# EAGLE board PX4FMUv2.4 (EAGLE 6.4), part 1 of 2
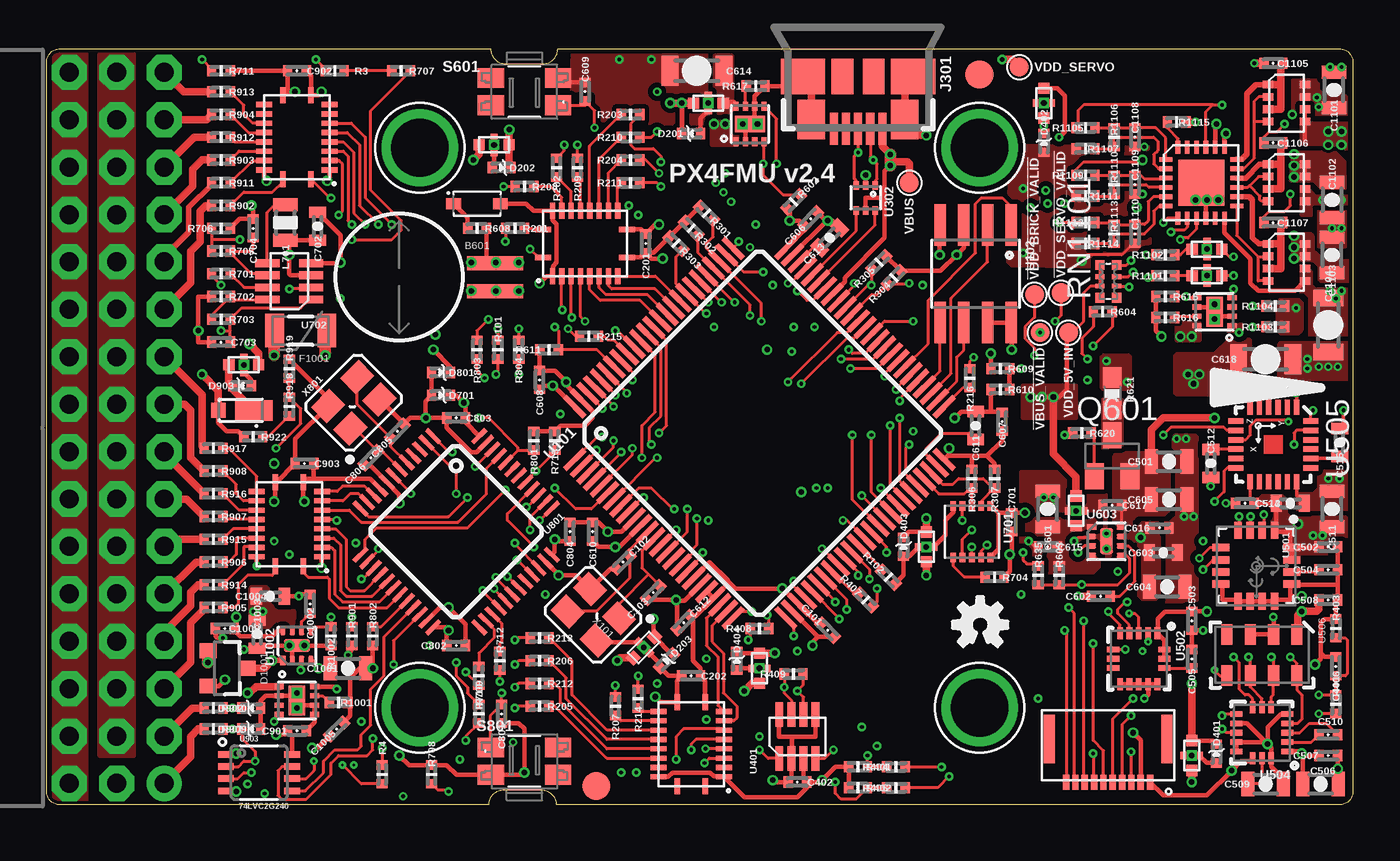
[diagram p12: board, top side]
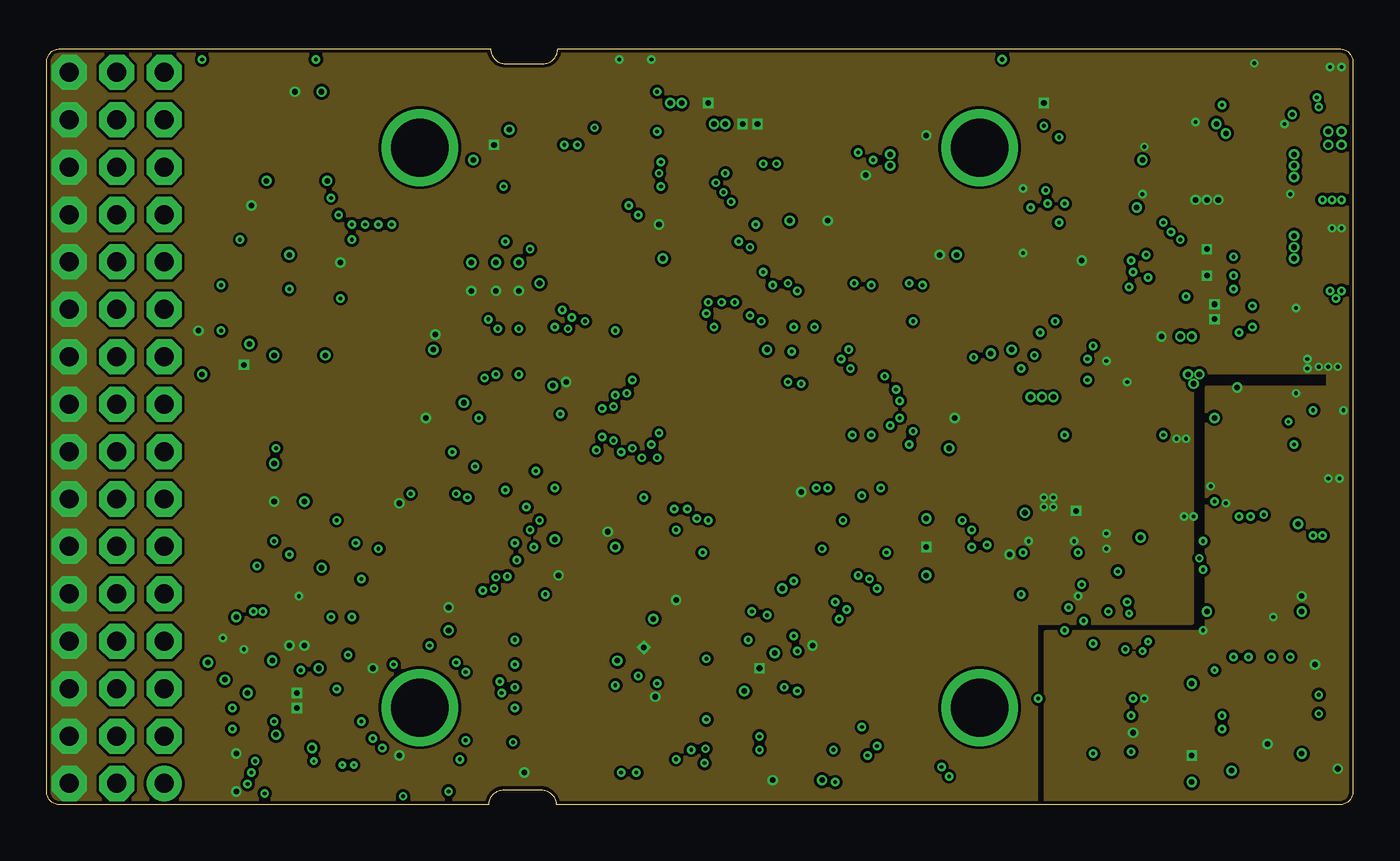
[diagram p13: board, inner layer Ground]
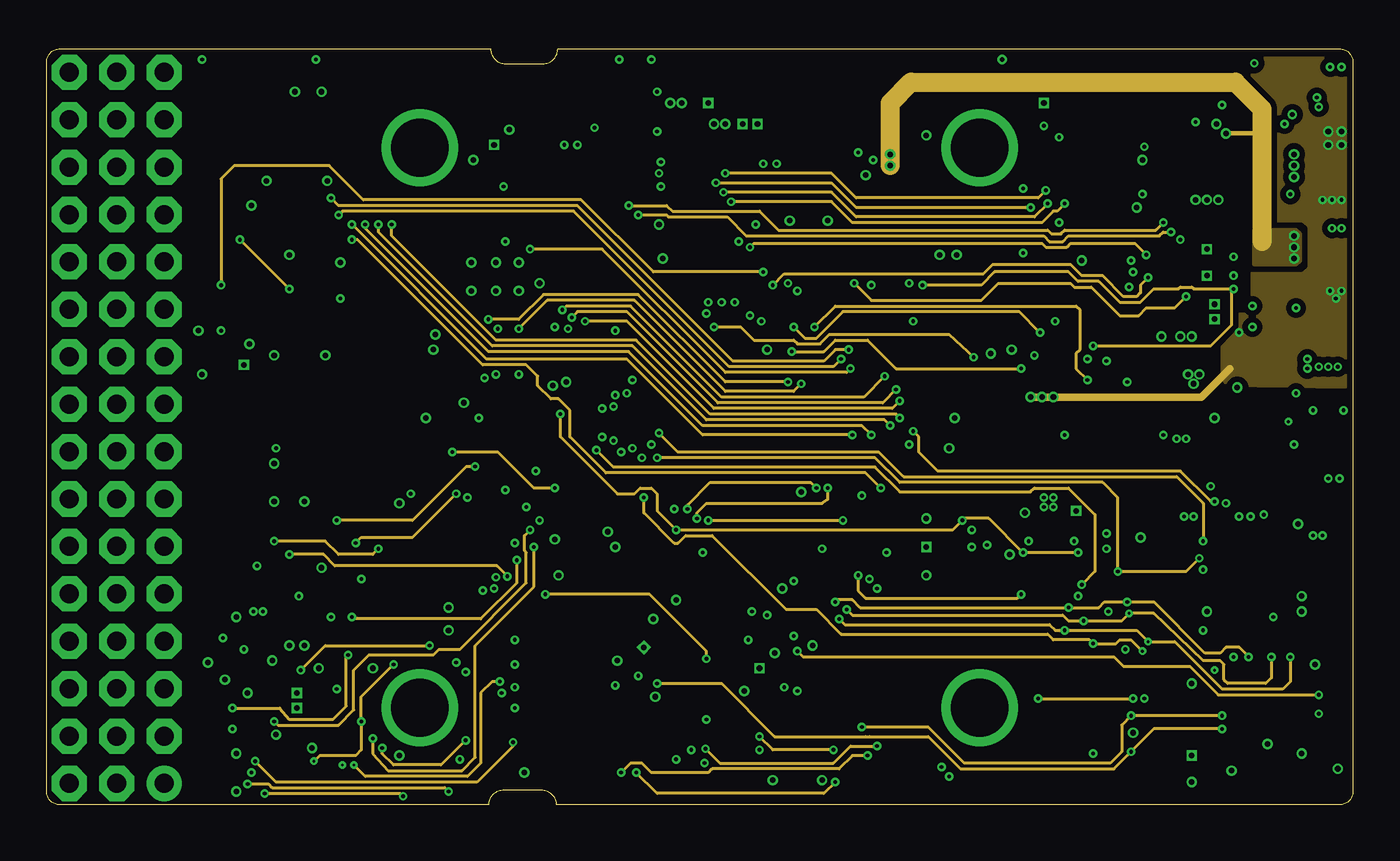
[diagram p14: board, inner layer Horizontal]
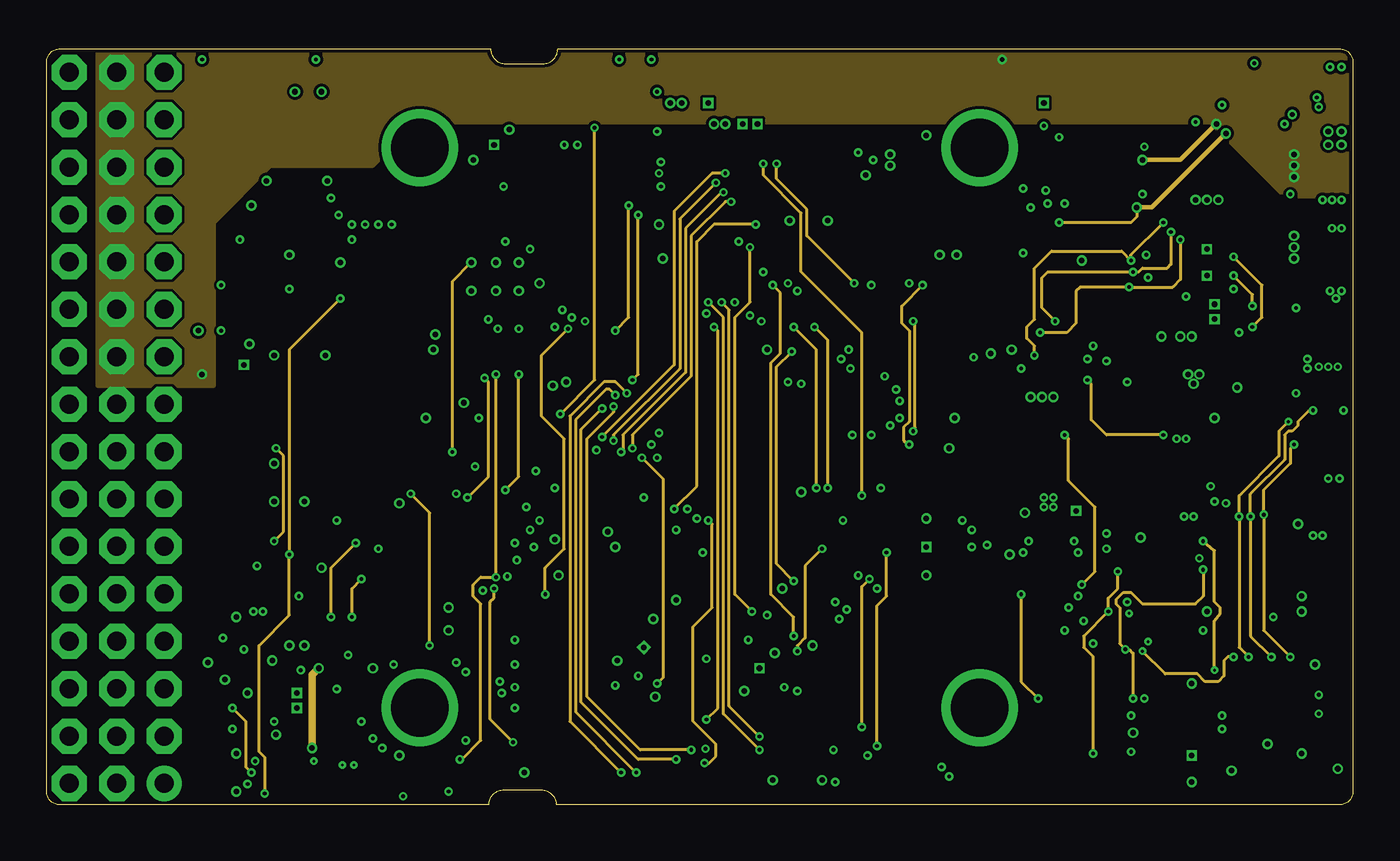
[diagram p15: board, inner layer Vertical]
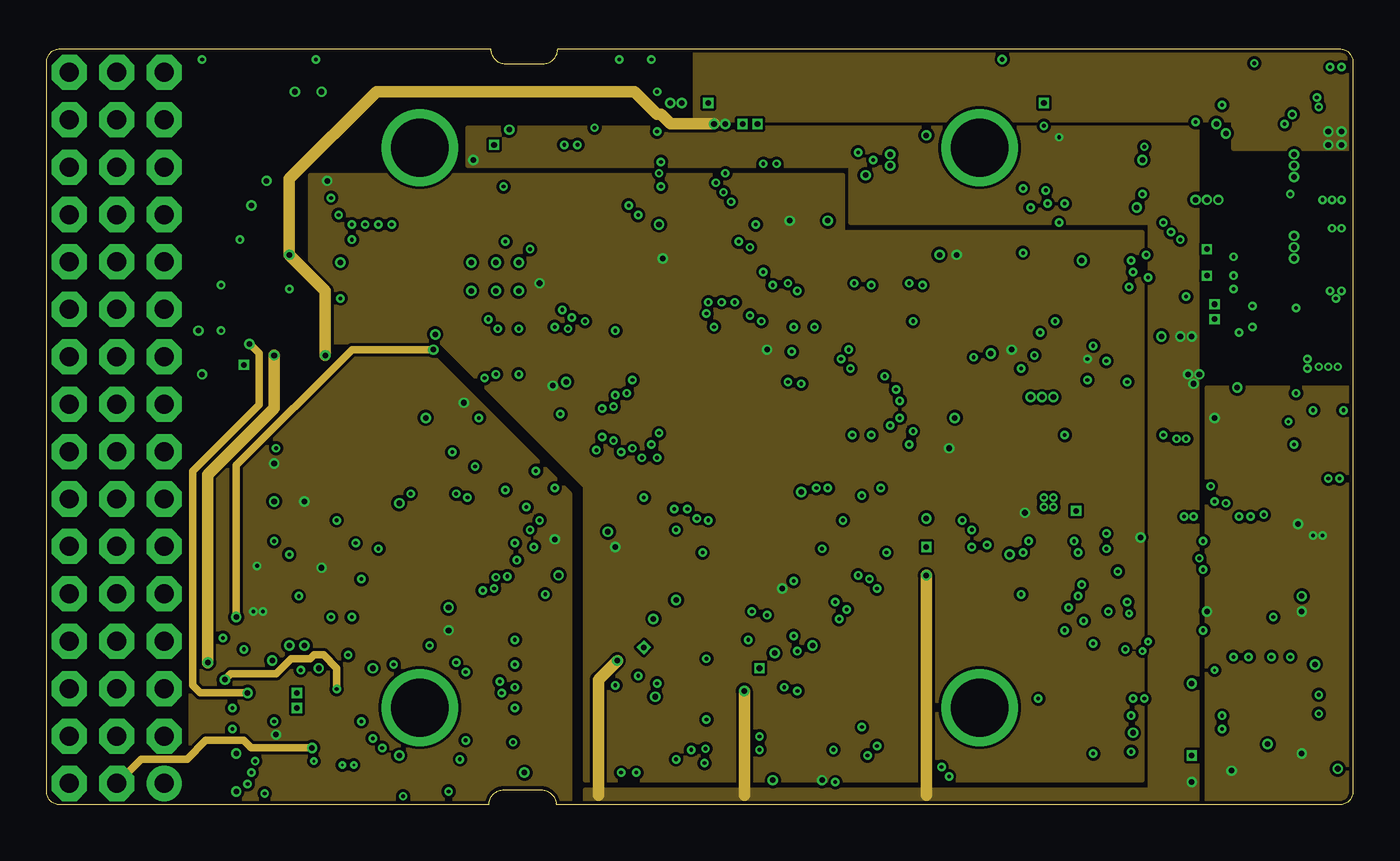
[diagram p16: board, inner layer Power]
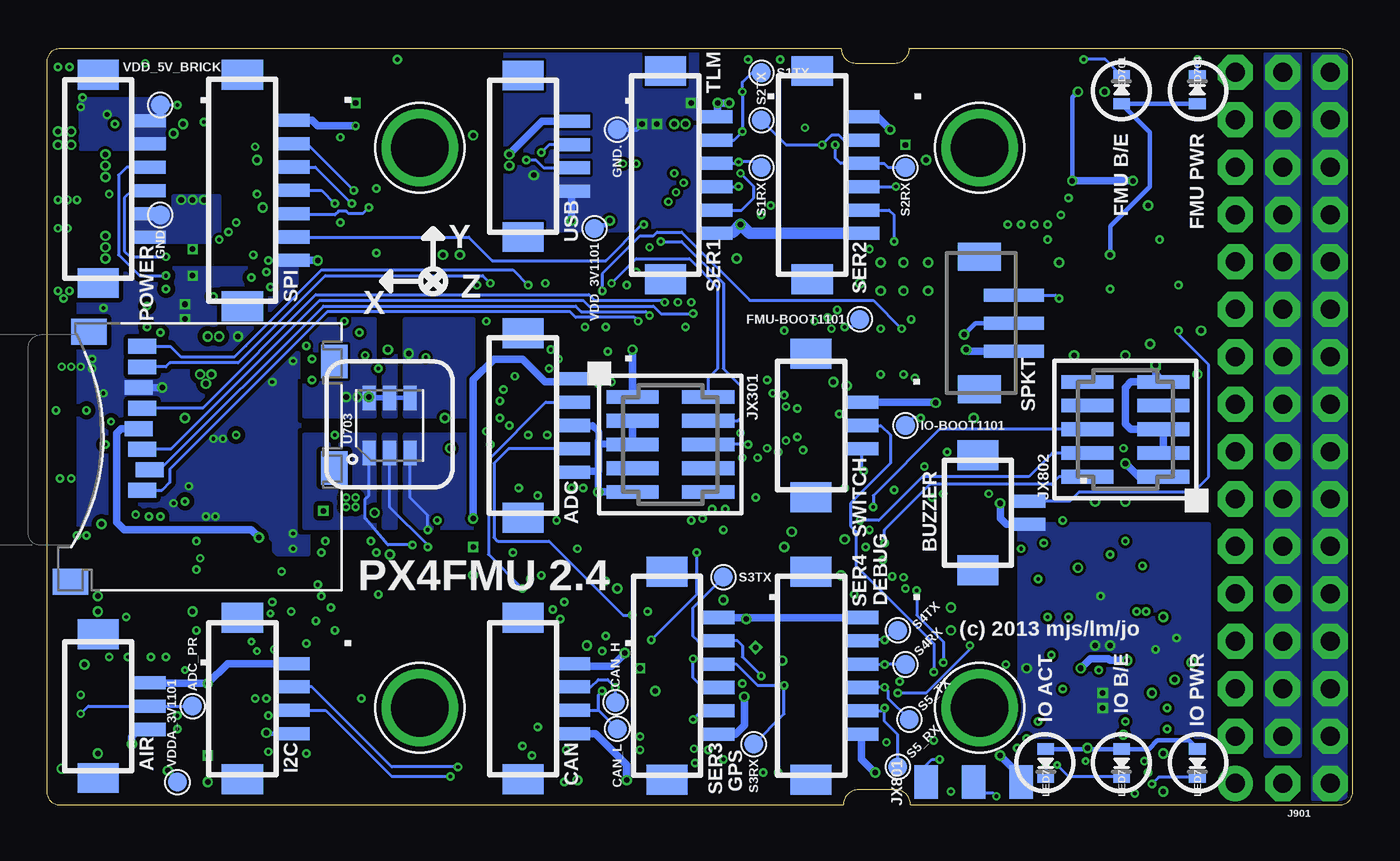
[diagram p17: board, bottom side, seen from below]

Size 70 x 40.5 mm. Coordinates in mm from the lower left corner, seen from the top.
Outline: 23.7,0 0.7,0 arc-90 0,0.7 0,39.8 arc-90 0.7,40.5 23.8,40.5 arc90 24.59,39.7 26.59,39.7 arc90 27.39,40.5 69.3,40.5 arc-90 70,39.8 70,0.7 arc-90 69.3,0 27.3,0 arc90 26.5,0.8 24.5,0.8 arc90 23.7,0
Copper layers (1*2*3*14*15*16): Top 0.035mm / dielectric 0.5mm / Ground 0.035mm / dielectric 0.15mm / Horizontal 0.035mm / dielectric 0.15mm / Vertical 0.035mm / dielectric 0.15mm / Power 0.035mm / dielectric 0.5mm / Bottom 0.035mm
Design rules "default *": minimum track width 0.15mm, minimum drill 0.2mm, track to track 5mil, track to pad 5mil, pad to pad 5mil, via to via 5mil, smd to smd 0mil, copper to edge 0.2mm, drill to drill 0.2mm, minimum pad ring 0.125mm, minimum via ring 0.125mm, stop-mask expansion 1mil, vias tented up to drill 0.31mm, thermal gap 8mil
Net classes: 0 signal: width 0.15 mm, drill 0.15 mm, clearance 0.152 mm; 1 power: width 0.15 mm, drill 0.2 mm, clearance 0.152 mm

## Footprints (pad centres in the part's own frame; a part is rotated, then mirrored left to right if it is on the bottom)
PAD.04X.04 = smd 1.016 x 1.016: P$1 0,0
MS621FE = smd 3 x 0.75: 1 5.15,0.75; 2 5.15,-0.75
0402-CAP = smd 0.5 x 0.6: P$1 -0.5,0; P$2 0.5,0
0805-CAP = smd 0.7 x 1.3: P$1 -0.95,0; P$2 0.95,0
0603-CAP = smd 0.6 x 0.9: P$1 -0.75,0; P$2 0.75,0
1206-CAP = smd 0.9 x 1.6: P$1 -1.45,0; P$2 1.45,0
MICROSMP = smd 0.8 x 0.8: ANODE 0.65,0 | smd 2 x 1.1: CATHODE -1.25,0
SOD323 = smd 0.8 x 0.6: A 1.25,0; C -1.25,0
0402-TVS = smd 0.5 x 0.6: A 0.5,0; C -0.5,0
SOT23-3 = smd 0.8 x 0.9: 1 -0.95,-1; 2 0.95,-1; 3 0,1.1
PTC-1206 = smd 1 x 1.8: 1 -1.4,0; 2 1.4,0
DF13C-6P-1.25V = smd 0.7 x 1.8: 1 -3.125,0.9; 2 -1.875,0.9; 3 -0.625,0.9; 4 0.625,0.9; 5 1.875,0.9; 6 3.125,0.9 | smd 1.6 x 2.2: M$0 5.575,-1.8; M$1 -5.575,-1.8
MOLEX-47346-0001 = smd 1.7 x 0.44: D+ 2.8,0; D- 2.8,0.65; GND 2.8,-1.3; ID 2.8,-0.65; VBUS 2.8,1.3 | smd 1.9 x 2.375: GND1 0,2.95; GND4 0,-2.95 | smd 2.1 x 1.475: GND2 2.3,2.5; GND3 2.3,-2.5 | smd 1.9 x 1.175: GND5 0,-0.838; GND6 0,0.838
DF13C-4P-1.25V = smd 0.7 x 1.8: 1 -1.875,0.9; 2 -0.625,0.9; 3 0.625,0.9; 4 1.875,0.9 | smd 1.6 x 2.2: M$0 4.325,-1.8; M$1 -4.325,-1.8
DF13C-3P-1.25V = smd 0.7 x 1.8: 1 -1.25,0.9; 2 0,0.9; 3 1.25,0.9 | smd 1.6 x 2.2: M$0 3.85,-1.8; M$1 -3.85,-1.8
DF13C-7P-1.25V = smd 0.7 x 1.8: 1 -3.75,0.9; 2 -2.5,0.9; 3 -1.25,0.9; 4 0,0.9; 5 1.25,0.9; 6 2.5,0.9; 7 3.75,0.9 | smd 1.6 x 2.2: M$0 6.2,-1.8; M$1 -6.2,-1.8
DF13C-5P-1.25V = smd 0.7 x 1.8: 1 -2.5,0.9; 2 -1.25,0.9; 3 0,0.9; 4 1.25,0.9; 5 2.5,0.9 | smd 1.6 x 2.2: M$0 4.95,-1.8; M$1 -4.95,-1.8
DF13C-2P-1.25V = smd 0.7 x 1.8: 1 -0.625,0.9; 2 0.625,0.9 | smd 1.6 x 2.2: M$0 3.075,-1.8; M$1 -3.075,-1.8
JST-ZH-SMT-VERTICAL = smd 0.7 x 3.2: P$1 -1.5,-1.75; P$2 0,-1.75; P$3 1.5,-1.75 | smd 1.5 x 2.3: P$4 3.55,0.1; P$5 -3.55,0.1
3X16RA = drill 1.016 pad 1.88: 1 2.54,19.05 | drill 1.016 pad 1.88 octagon: 2 0,19.05; 3 -2.54,19.05; 4 2.54,16.51; 5 0,16.51; 6 -2.54,16.51; 7 2.54,13.97; 8 0,13.97; 9 -2.54,13.97; 10 2.54,11.43; 11 0,11.43; 12 -2.54,11.43; 13 2.54,8.89; 14 0,8.89; 15 -2.54,8.89; 16 2.54,6.35; 17 0,6.35; 18 -2.54,6.35; 19 2.54,3.81; 20 0,3.81; 21 -2.54,3.81; 22 2.54,1.27; 23 0,1.27; 24 -2.54,1.27; 25 2.54,-1.27; 26 0,-1.27; 27 -2.54,-1.27; 28 2.54,-3.81; 29 0,-3.81; 30 -2.54,-3.81; 31 2.54,-6.35; 32 0,-6.35; 33 -2.54,-6.35; 34 2.54,-8.89; 35 0,-8.89; 36 -2.54,-8.89; 37 2.54,-11.43; 38 0,-11.43; 39 -2.54,-11.43; 40 2.54,-13.97; 41 0,-13.97; 42 -2.54,-13.97; 43 2.54,-16.51; 44 0,-16.51; 45 -2.54,-16.51; 46 2.54,-19.05; 47 0,-19.05; 48 -2.54,-19.05
FIDUCIAL-1.5X3 = smd 1.5 x 1.5: 1 0,0
FTSH-105-01-XXX-DV-K = smd 0.737 x 2.794: 1 -2.54,-2.032; 2 -2.54,2.032; 3 -1.27,-2.032; 4 -1.27,2.032; 5 0,-2.032; 6 0,2.032; 7 1.27,-2.032; 8 1.27,2.032; 9 2.54,-2.032; 10 2.54,2.032
HEADER_3X01_SMD_H_BOARD_EDGE_SHORT = smd 1.27 x 1.778: 1 -2.54,0; 2 0,0; 3 2.54,0
KYOCERA-KNH16-DA = smd 0.6 x 0.6: P$1 -0.8,0; P$2 0.8,0 | smd 0.4 x 0.4: P$3 0,-0.4; P$4 0,0.4 | drill 0.3 pad 0.4 square: P$5 0,0
0805-IND = smd 0.7 x 1.3: P$1 -0.95,0; P$2 0.95,0
0603-LED = smd 0.6 x 0.9: A 0.75,0; C -0.75,0
MOUNT-HOLE3.1 = drill 3.1 pad 4.1: P$1 0,0
SOT23-BEC = smd 1 x 1.4: B -0.95,-1.1; C 0,1.1; E 0.95,-1.1
0402-RES = smd 0.5 x 0.6: P$1 -0.5,0; P$2 0.5,0
0603-RES = smd 1.1 x 1: 1 -0.85,0; 2 0.85,0
EXB28V = smd 0.525 x 0.5: 1 -0.875,-0.45; 4 0.875,-0.45; 5 0.875,0.45; 8 -0.875,0.45 | smd 0.25 x 0.5: 2 -0.25,-0.45; 3 0.25,-0.45; 6 0.25,0.45; 7 -0.25,0.45
EVQP7J01K = smd 1.4 x 1.05: A1 -1.8,0.725; A2 1.8,0.725; B3 -1.8,-0.725; B4 1.8,-0.725
TQFP100 = smd 1.5 x 0.29: 1 -8,6; 2 -8,5.5; 3 -8,5; 4 -8,4.5; 5 -8,4; 6 -8,3.5; 7 -8,3; 8 -8,2.5; 9 -8,2; 10 -8,1.5; 11 -8,1; 12 -8,0.5; 13 -8,0; 14 -8,-0.5; 15 -8,-1; 16 -8,-1.5; 17 -8,-2; 18 -8,-2.5; 19 -8,-3; 20 -8,-3.5; 21 -8,-4; 22 -8,-4.5; 23 -8,-5; 24 -8,-5.5; 25 -8,-6; 51 8,-6; 52 8,-5.5; 53 8,-5; 54 8,-4.5; 55 8,-4; 56 8,-3.5; 57 8,-3; 58 8,-2.5; 59 8,-2; 60 8,-1.5; 61 8,-1; 62 8,-0.5; 63 8,0; 64 8,0.5; 65 8,1; 66 8,1.5; 67 8,2; 68 8,2.5; 69 8,3; 70 8,3.5; 71 8,4; 72 8,4.5; 73 8,5; 74 8,5.5; 75 8,6 | smd 0.29 x 1.5: 26 -6,-8; 27 -5.5,-8; 28 -5,-8; 29 -4.5,-8; 30 -4,-8; 31 -3.5,-8; 32 -3,-8; 33 -2.5,-8; 34 -2,-8; 35 -1.5,-8; 36 -1,-8; 37 -0.5,-8; 38 0,-8; 39 0.5,-8; 40 1,-8; 41 1.5,-8; 42 2,-8; 43 2.5,-8; 44 3,-8; 45 3.5,-8; 46 4,-8; 47 4.5,-8; 48 5,-8; 49 5.5,-8; 50 6,-8; 76 6,8; 77 5.5,8; 78 5,8; 79 4.5,8; 80 4,8; 81 3.5,8; 82 3,8; 83 2.5,8; 84 2,8; 85 1.5,8; 86 1,8; 87 0.5,8; 88 0,8; 89 -0.5,8; 90 -1,8; 91 -1.5,8; 92 -2,8; 93 -2.5,8; 94 -3,8; 95 -3.5,8; 96 -4,8; 97 -4.5,8; 98 -5,8; 99 -5.5,8; 100 -6,8
SO08 = smd 0.61 x 2.21: 1 -1.905,-2.616; 2 -0.635,-2.616; 3 0.635,-2.616; 4 1.905,-2.616; 5 1.905,2.616; 6 0.635,2.616; 7 -0.635,2.616; 8 -1.905,2.616
QFN20-RGY = smd 0.28 x 0.85: 1 -0.75,2.25; 10 -0.75,-2.25; 11 0.75,-2.25; 20 0.75,2.25 | smd 0.85 x 0.28: 2 -1.75,1.75; 3 -1.75,1.25; 4 -1.75,0.75; 5 -1.75,0.25; 6 -1.75,-0.25; 7 -1.75,-0.75; 8 -1.75,-1.25; 9 -1.75,-1.75; 12 1.75,-1.75; 13 1.75,-1.25; 14 1.75,-0.75; 15 1.75,-0.25; 16 1.75,0.25; 17 1.75,0.75; 18 1.75,1.25; 19 1.75,1.75
MICROSD = smd 0.8 x 1.5: 1 -1.94,2.7; 2 -0.84,2.3; 3 0.26,2.7; 4 1.36,2.9; 5 2.46,2.7; 6 3.56,2.9; 7 4.66,2.7; 8 5.76,2.7 | smd 1.4 x 1.9: NC -6.85,6.55; NC3 6.55,5.55 | smd 1.8 x 1.4: NC1 -0.75,-7.6; NC2 4.95,-7.6
SOT563-6 = smd 0.3 x 0.45: 1 -0.5,-0.675; 2 0,-0.675; 3 0.5,-0.675; 4 0.5,0.675; 5 0,0.675; 6 -0.5,0.675
SOT23-8 = smd 0.42 x 1.3: 1 -0.975,-1.175; 2 -0.325,-1.175; 3 0.325,-1.175; 4 0.975,-1.175; 5 0.975,1.175; 6 0.325,1.175; 7 -0.325,1.175; 8 -0.975,1.175
L3G4200DH-MAN = smd 0.9 x 0.4: 1 -1.9,0.975; 2 -1.9,0.325; 3 -1.9,-0.325; 4 -1.9,-0.975; 9 1.9,-0.975; 10 1.9,-0.325; 11 1.9,0.325; 12 1.9,0.975 | smd 0.4 x 0.9: 5 -0.975,-1.9; 6 -0.325,-1.9; 7 0.325,-1.9; 8 0.975,-1.9; 13 0.975,1.9; 14 0.325,1.9; 15 -0.325,1.9; 16 -0.975,1.9
LGA-16L = smd 0.65 x 0.3: 1 -1.37,1; 2 -1.37,0.5; 3 -1.37,0; 4 -1.37,-0.5; 5 -1.37,-1; 9 1.37,-1; 10 1.37,-0.5; 11 1.37,0; 12 1.37,0.5; 13 1.37,1 | smd 0.3 x 0.65: 6 -0.5,-1.37; 7 0,-1.37; 8 0.5,-1.37; 14 0.5,1.37; 15 0,1.37; 16 -0.5,1.37
QFN-24 = smd 0.8 x 0.29: 1 -2,1.25; 2 -2,0.75; 3 -2,0.25; 4 -2,-0.25; 5 -2,-0.75; 6 -2,-1.25; 13 2,-1.25; 14 2,-0.75; 15 2,-0.25; 16 2,0.25; 17 2,0.75; 18 2,1.25 | smd 0.29 x 0.8: 7 -1.25,-2; 8 -0.75,-2; 9 -0.25,-2; 10 0.25,-2; 11 0.75,-2; 12 1.25,-2; 19 1.25,2; 20 0.75,2; 21 0.25,2; 22 -0.25,2; 23 -0.75,2; 24 -1.25,2
MS5611-01BA = smd 1.1 x 0.6: 1 -1.1,1.875; 2 -1.1,0.625; 3 -1.1,-0.625; 4 -1.1,-1.875; 5 1.1,-1.875; 6 1.1,-0.625; 7 1.1,0.625; 8 1.1,1.875
QFN8-DSG = smd 0.28 x 0.5: 1 -0.75,-0.95; 2 -0.25,-0.95; 3 0.25,-0.95; 4 0.75,-0.95; 5 0.75,0.95; 6 0.25,0.95; 7 -0.25,0.95; 8 -0.75,0.95 | smd 1.6 x 0.9: GND 0,0 | drill 0.3 square: P$2 -0.4,0; P$3 0.4,0
MLF-8-EPAD = smd 0.5 x 0.3: 1 -0.8,0.75; 2 -0.8,0.25; 3 -0.8,-0.25; 4 -0.8,-0.75; 5 0.8,-0.75; 6 0.8,-0.25; 7 0.8,0.25; 8 0.8,0.75 | smd 0.7 x 1.4: GND 0,0
SON10 = smd 0.32 x 0.5: 1 -1,-1.375; 2 -0.5,-1.375; 3 0,-1.375; 4 0.5,-1.375; 5 1,-1.375; 6 1,1.375; 7 0.5,1.375; 8 0,1.375; 9 -0.5,1.375; 10 -1,1.375
6-PLCC = smd 1.3 x 0.7: A1 1.475,1.1; A2 1.475,0; A3 1.475,-1.1; C1 -1.475,1.1; C2 -1.475,0; C3 -1.475,-1.1
TQFP48 = smd 0.24 x 1: 1 -2.75,-4.5; 2 -2.25,-4.5; 3 -1.75,-4.5; 4 -1.25,-4.5; 5 -0.75,-4.5; 6 -0.25,-4.5; 7 0.25,-4.5; 8 0.75,-4.5; 9 1.25,-4.5; 10 1.75,-4.5; 11 2.25,-4.5; 12 2.75,-4.5; 25 2.75,4.5; 26 2.25,4.5; 27 1.75,4.5; 28 1.25,4.5; 29 0.75,4.5; 30 0.25,4.5; 31 -0.25,4.5; 32 -0.75,4.5; 33 -1.25,4.5; 34 -1.75,4.5; 35 -2.25,4.5; 36 -2.75,4.5 | smd 1 x 0.24: 13 4.5,-2.75; 14 4.5,-2.25; 15 4.5,-1.75; 16 4.5,-1.25; 17 4.5,-0.75; 18 4.5,-0.25; 19 4.5,0.25; 20 4.5,0.75; 21 4.5,1.25; 22 4.5,1.75; 23 4.5,2.25; 24 4.5,2.75; 37 -4.5,2.75; 38 -4.5,2.25; 39 -4.5,1.75; 40 -4.5,1.25; 41 -4.5,0.75; 42 -4.5,0.25; 43 -4.5,-0.25; 44 -4.5,-0.75; 45 -4.5,-1.25; 46 -4.5,-1.75; 47 -4.5,-2.25; 48 -4.5,-2.75
TSSOP8_SOT505-2 = smd 0.35 x 0.85: 1 -0.975,-1.775; 2 -0.325,-1.775; 3 0.325,-1.775; 4 0.975,-1.775; 5 0.975,1.775; 6 0.325,1.775; 7 -0.325,1.775; 8 -0.975,1.775
MO-220 = smd 0.7 x 0.25: P$1 -1.9,1.25; P$2 -1.9,0.75; P$3 -1.9,0.25; P$4 -1.9,-0.25; P$5 -1.9,-0.75; P$6 -1.9,-1.25; P$13 1.9,-1.25; P$14 1.9,-0.75; P$15 1.9,-0.25; P$16 1.9,0.25; P$17 1.9,0.75; P$18 1.9,1.25 | smd 0.25 x 0.7: P$7 -1.25,-1.9; P$8 -0.75,-1.9; P$9 -0.25,-1.9; P$10 0.25,-1.9; P$11 0.75,-1.9; P$12 1.25,-1.9; P$19 1.25,1.9; P$20 0.75,1.9; P$21 0.25,1.9; P$22 -0.25,1.9; P$23 -0.75,1.9; P$24 -1.25,1.9 | smd 2.45 x 2.45: P$25 0,0
1206-8 = smd 0.406 x 0.559: P$1 -0.991,-0.991; P$2 -0.33,-0.991; P$3 0.33,-0.991; P$4 0.991,-0.991; P$5 0.991,0.991; P$6 0.33,0.991; P$7 -0.33,0.991; P$8 -0.991,0.991
OSCILLATOR-3.2X2.5 = smd 1.4 x 1.2: 1 -1.1,-0.85; 2 1.1,-0.85; 3 1.1,0.85; 4 -1.1,0.85
51281-1094 = smd 0.34 x 0.8: 1 0,0; 2 0.5,0; 3 1,0; 4 1.5,0; 5 2,0; 6 2.5,0; 7 3,0; 8 3.5,0; 9 4,0; 10 4.5,0 | smd 0.6 x 2.6: P$11 -0.9,-2.3; P$12 5.4,-2.3

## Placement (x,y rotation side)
!VBUS_VALID  PAD.04  [PAD.04X.04]  53.24,25.3 270 top
!VDD_BRICK_VALID  PAD.04  [PAD.04X.04]  52.93,27.33 90 top
!VDD_SERVO_VALID  PAD.04  [PAD.04X.04]  54.36,27.43 90 top
ADC_PR  PAD.04  [PAD.04X.04]  62.18,5.28 270 bottom
B601  MS621FE  [MS621FE]  18.89,28.27 0 top
C101  0u1  [0402-CAP]  41.86,9.35 315 top
C102  8p  [0402-CAP]  30.89,13 225 top
C103  8p  [0402-CAP]  32.51,11.38 45 top
C201  0u1  [0402-CAP]  32.11,30.07 90 top
C202  0u1  [0402-CAP]  34.54,6.91 180 top
C401  0u1  [0402-CAP]  69.09,7.42 90 top
C402  0u1  [0402-CAP]  40.23,1.22 180 top
C501  10u/10V  [0805-CAP]  60.15,18.39 0 top
C502  0u1  [0402-CAP]  68.68,13.82 0 top
C503  0u1  [0402-CAP]  61.37,9.86 270 top
C504  10n  [0402-CAP]  68.68,12.6 0 top
C505  10n  [0402-CAP]  61.37,7.82 90 top
C506  10u/10V  [0805-CAP]  68.28,1.12 0 top
C507  0u1  [0402-CAP]  68.68,2.64 0 top
C508  0u1  [0402-CAP]  68.68,10.97 0 top
C509  10u/10V  [0805-CAP]  65.33,1.12 0 top
C510  0u47  [0402-CAP]  68.68,3.76 0 top
C511  10u/10V  [0805-CAP]  68.88,15.85 90 top
C512  2u2  [0603-CAP]  62.38,18.29 270 top
C513  2u2  [0603-CAP]  66.65,16.15 0 top
C514  0u1  [0402-CAP]  64.21,16.15 180 top
C515  0u01  [0603-CAP]  69.29,19.41 90 top
C601  10u/25V  [0805-CAP]  53.64,15.85 90 top
C602  10n  [0402-CAP]  56.49,11.18 0 top
C603  1u  [0603-CAP]  59.84,13.51 0 top
C604  22u/25V  [0805-CAP]  60.05,11.68 0 top
C605  22u/25V  [0805-CAP]  60.15,16.36 0 top
C606  0u1  [0402-CAP]  40.94,31.39 45 top
C607  0u1  [0402-CAP]  51.21,20.52 90 top
C608  0u1  [0402-CAP]  26.42,22.76 90 top
C609  0u1  [0402-CAP]  28.85,38.2 270 top
C610  0u1  [0402-CAP]  29.26,14.63 90 top
C611  2u2  [0603-CAP]  49.78,20.32 90 top
C612  0u1  [0402-CAP]  34.14,9.75 225 top
C613  2u2  [0603-CAP]  41.96,30.38 45 top
C614  100u  [1206-CAP]  34.85,39.32 180 top
C615  0u1  [0402-CAP]  53.64,13.82 180 top
C616  0u1  [0402-CAP]  59.64,14.83 0 top
C617  0u1  [0402-CAP]  57.1,16.05 180 top
C618  100u  [1206-CAP]  65.33,23.88 0 top
C701  0u1  [0402-CAP]  51.71,15.14 270 top
C702  1u0  [0603-CAP]  14.53,30.99 90 top
C703  5n6  [0402-CAP]  9.35,24.79 180 top
C704  0u47  [0402-CAP]  11.07,30.89 90 top
C801  0u1  [0402-CAP]  24.38,4.88 90 top
C802  0u1  [0402-CAP]  21.95,8.53 0 top
C803  0u1  [0402-CAP]  21.95,20.73 180 top
C804  0u1  [0402-CAP]  28.04,14.63 90 top
C805  8p  [0402-CAP]  18.8,20.02 45 top
C806  8p  [0402-CAP]  17.37,18.59 45 top
C901  0u1  [0402-CAP]  13.41,3.96 0 top
C902  0u1  [0402-CAP]  13.41,39.32 180 top
C903  0u1  [0402-CAP]  13.82,18.29 180 top
C1001  10u/25V  [0805-CAP]  16.15,7.32 0 top
C1002  10n  [0402-CAP]  14.12,10.77 90 top
C1003  1u0  [0603-CAP]  11.28,9.14 270 top
C1004  10u  [0603-CAP]  11.99,11.18 0 top
C1005  0u1F  [0402-CAP]  15.54,4.06 45 top
C1008  2u2  [0402-CAP]  9.55,9.45 180 top
C1101  22u/25V  [0805-CAP]  68.99,38.3 90 top
C1102  22u/25V  [0805-CAP]  68.88,32.41 270 top
C1103  22u/25V  [0805-CAP]  68.88,29.46 90 top
C1104  100u  [1206-CAP]  68.68,25.7 270 top
C1105  0u1  [0402-CAP]  65.74,39.73 180 top
C1106  0u1  [0402-CAP]  65.74,35.46 180 top
C1107  0u1  [0402-CAP]  65.74,31.19 180 top
C1108  1000p/25V  [0402-CAP]  58.32,35.76 270 top
C1109  1000p/25V  [0402-CAP]  58.32,33.22 270 top
C1110  1000p/25V  [0402-CAP]  58.32,30.58 270 top
CAN_H  PAD.04  [PAD.04X.04]  39.52,5.49 90 bottom
CAN_L  PAD.04  [PAD.04X.04]  39.42,4.06 270 bottom
D1  MSS1P4-M3  [MICROSMP]  9.86,21.13 180 top
D2  RB751V40T1G  [SOD323]  23.06,32.21 0 top
D201  PESD0402-140  [0402-TVS]  34.54,35.97 0 top
D202  PESD0402-140  [0402-TVS]  24.38,34.14 180 top
D203  PESD0402-140  [0402-TVS]  33.22,7.72 225 top
D401  PESD0402-140  [0402-TVS]  62.69,2.74 270 top
D402  PESD0402-140  [0402-TVS]  53.44,35.46 270 top
D403  PESD0402-140  [0402-TVS]  45.92,13.82 270 top
D404  PESD0402-140  [0402-TVS]  36.98,7.72 270 top
D701  PESD0402-140  [0402-TVS]  21.13,21.95 180 top
D801  PESD0402-140  [0402-TVS]  21.13,23.16 180 top
D901  PESD0402-140  [0402-TVS]  10.97,4.06 0 top
D902  PESD0402-140  [0402-TVS]  10.97,5.18 0 top
D903  PESD0402-140  [0402-TVS]  10.46,22.45 0 top
D1001  PMEG2005CT  [SOT23-3]  9.65,7.32 270 top
F1001  0ZCA0035FF2G  [PTC-1206]  13.61,25.4 180 top
FMU-BOOT1101  PAD.04  [PAD.04X.04]  26.42,26.01 0 bottom
GND  PAD.04  [PAD.04X.04]  63.91,31.6 270 bottom
GND.  PAD.04  [PAD.04X.04]  39.42,36.17 0 bottom
IO-BOOT1101  PAD.04  [PAD.04X.04]  23.98,20.32 0 bottom
J201  DF13C-6P-1.25V  [DF13C-6P-1.25V]  35.04,33.74 270 bottom
J202  DF13C-6P-1.25V  [DF13C-6P-1.25V]  27.17,33.74 270 bottom
J203  DF13C-6P-1.25V  [DF13C-6P-1.25V]  34.95,6.91 270 bottom
J204  DF13C-6P-1.25V  [DF13C-6P-1.25V]  27.23,6.91 270 bottom
J301  47346-0001  [MOLEX-47346-0001]  43.48,39.01 270 top
J302  DF13C-4P-1.25V  [DF13C-4P-1.25V]  42.67,34.75 270 bottom
J401  DF13C-4P-1.25V  [DF13C-4P-1.25V]  57.71,5.69 270 bottom
J402  DF13C-3P-1.25V  [DF13C-3P-1.25V]  65.43,5.28 270 bottom
J403  DF13C-7P-1.25V  [DF13C-7P-1.25V]  57.71,32.92 270 bottom
J404  DF13C-5P-1.25V  [DF13C-5P-1.25V]  42.67,20.32 270 bottom
J405  DF13C-4P-1.25V  [DF13C-4P-1.25V]  42.67,5.69 270 bottom
J601  DF13C-6P-1.25V  [DF13C-6P-1.25V]  65.43,33.53 270 bottom
J701  DF13C-2P-1.25V  [DF13C-2P-1.25V]  18.29,15.65 270 bottom
J702  DF13C-3P-1.25V  [DF13C-3P-1.25V]  27.23,20.32 270 bottom
J801  JST-ZH-3  [JST-ZH-SMT-VERTICAL]  19.91,25.81 90 bottom
J901  [3X16RA]  3.76,20.19 180 bottom
JP1  FIDUCIAL1.5X3  [FIDUCIAL-1.5X3]  49.99,39.12 0 top
JP2  FIDUCIAL1.5X3  [FIDUCIAL-1.5X3]  29.46,1.02 0 top
JX301  ARM_MINI_JTAG-SMT  [FTSH-105-01-XXX-DV-K]  36.58,19.3 270 bottom
JX801  HEADER-3X1BOARDEDGE-SHORT  [HEADER_3X01_SMD_H_BOARD_EDGE_SHORT]  20.32,1.22 0 bottom
JX802  ARM_MINI_JTAG-SMT  [FTSH-105-01-XXX-DV-K]  12.19,20.12 90 bottom
L201  KNH16C104DA5TS  [KYOCERA-KNH16-DA]  35.46,37.59 180 top
L202  KNH16C104DA5TS  [KYOCERA-KNH16-DA]  23.98,35.36 0 top
L203  KNH16C104DA5TS  [KYOCERA-KNH16-DA]  32,8.43 45 top
L401  KNH16C104DA5TS  [KYOCERA-KNH16-DA]  61.37,2.64 90 top
L402  KNH16C104DA5TS  [KYOCERA-KNH16-DA]  53.44,37.59 270 top
L403  KNH16C104DA5TS  [KYOCERA-KNH16-DA]  38.2,7.32 90 top
L404  KNH16C104DA5TS  [KYOCERA-KNH16-DA]  47.14,13.82 90 top
L603  KNH16C104DA5TS  [KYOCERA-KNH16-DA]  55.17,15.75 270 top
L701  47uH  [0805-IND]  12.8,31.19 90 top
L901  KNH16C104DA5TS  [KYOCERA-KNH16-DA]  10.57,23.57 0 top
L1101  KNH16C104DA5TS  [KYOCERA-KNH16-DA]  62.18,28.35 180 top
L1102  KNH16C104DA5TS  [KYOCERA-KNH16-DA]  62.18,29.77 180 top
LED701  AMBER  [0603-LED]  12.4,38.3 270 bottom
LED702  GREEN  [0603-LED]  8.33,2.24 90 bottom
LED703  AMBER  [0603-LED]  12.4,2.24 90 bottom
LED704  GREEN  [0603-LED]  8.33,38.3 270 bottom
LED705  BLUE  [0603-LED]  16.46,2.24 90 bottom
M3_MOUNT1101  MOUNT-HOLE3.1MM  [MOUNT-HOLE3.1]  20,35.2 0 top
M3_MOUNT1102  MOUNT-HOLE3.1MM  [MOUNT-HOLE3.1]  50,5.2 0 top
M3_MOUNT1103  MOUNT-HOLE3.1MM  [MOUNT-HOLE3.1]  50,35.2 0 top
M3_MOUNT1104  MOUNT-HOLE3.1MM  [MOUNT-HOLE3.1]  20,5.2 0 top
OSHW_LOGO  OSHW-LOGOS  [OSHW-LOGO-S]  50.03,9.65 0 top
Q601  MMBT3906LT1SMD  [SOT23-BEC]  57.1,18.69 0 top
R3  220R  [0402-RES]  15.44,39.32 180 top
R4  220R  [0402-RES]  17.98,1.63 270 top
R101  470R  [0402-RES]  24.18,24.38 270 top
R102  10K  [0402-RES]  45.11,12.19 315 top
R201  120R  [0402-RES]  25.1,30.89 180 top
R202  120R  [0402-RES]  27.33,34.14 90 top
R203  120R  [0402-RES]  31.29,36.98 0 top
R204  120R  [0402-RES]  31.29,34.54 0 top
R205  120R  [0402-RES]  26.42,5.28 180 top
R206  120R  [0402-RES]  26.42,7.72 180 top
R207  120R  [0402-RES]  30.48,5.28 90 top
R208  120R  [0402-RES]  25.6,33.12 180 top
R209  120R  [0402-RES]  28.45,34.14 90 top
R210  120R  [0402-RES]  31.29,35.76 0 top
R211  120R  [0402-RES]  31.29,33.32 0 top
R212  120R  [0402-RES]  26.42,6.5 180 top
R213  120R  [0402-RES]  26.42,8.94 180 top
R214  120R  [0402-RES]  31.7,5.69 90 top
R215  120R  [0402-RES]  29.06,25.1 180 top
R216  120R  [0402-RES]  49.48,22.86 90 top
R301  100K  [0402-RES]  35.36,31.7 135 top
R302  100K  [0402-RES]  34.54,30.89 135 top
R303  100K  [0402-RES]  33.73,30.07 135 top
R304  100K  [0402-RES]  45.42,28.24 45 top
R305  100K  [0402-RES]  44.6,29.06 45 top
R306  1K5  [0402-RES]  49.58,17.48 90 top
R307  1K5  [0402-RES]  50.8,17.48 90 top
R401  1K5  [0402-RES]  43.48,2.03 180 top
R402  1K5  [0402-RES]  43.48,0.91 180 top
R403  10K/0.1%  [0402-RES]  69.09,9.45 270 top
R404  120R  [0402-RES]  45.52,2.03 0 top
R405  120R  [0402-RES]  45.52,0.91 0 top
R406  10K/0.1%  [0402-RES]  69.09,5.38 270 top
R407  10K/0.1%  [0402-RES]  43.89,10.97 315 top
R408  10K/0.1%  [0402-RES]  38.2,9.45 0 top
R409  120R  [0402-RES]  40.03,7.01 0 top
R602  1M  [0402-RES]  40.03,32.31 225 top
R603  10k  [0402-RES]  54.25,12.29 270 top
R604  1M  [0402-RES]  56.59,26.42 180 top
R608  1K  [0402-RES]  23.06,30.89 180 top
R609  10K/0.1%  [0402-RES]  51.1,23.37 180 top
R610  10K/0.1%  [0402-RES]  51.1,22.25 180 top
R611  10K  [0402-RES]  26.92,24.38 0 top
R615  10K  [0402-RES]  59.94,27.23 180 top
R616  25K5  [0402-RES]  59.94,26.11 180 top
R617  16K5  [0402-RES]  38,38.51 0 top
R620  1k8  [0402-RES]  55.47,19.91 180 top
R621  10R  [0603-RES]  57.1,22.05 270 top
R635  DNP / 10k  [0402-RES]  53.14,12.29 270 top
R701  9K09  [0402-RES]  9.35,28.45 180 top
R702  10K  [0402-RES]  9.35,27.23 180 top
R703  100K  [0402-RES]  9.35,26.01 180 top
R704  10K  [0402-RES]  50.8,12.19 180 top
R705  453K  [0402-RES]  9.35,29.67 180 top
R706  16K5  [0402-RES]  9.35,30.89 0 top
R707  220R  [0402-RES]  19,39.32 180 top
R708  220R  [0402-RES]  20.62,1.63 270 top
R709  220R  [0402-RES]  23.16,4.88 270 top
R710  68R  [0402-RES]  23.16,6.91 90 top
R711  220R  [0402-RES]  9.35,39.32 180 top
R712  220R  [0402-RES]  24.28,7.72 270 top
R713  1K5  [0402-RES]  27.23,19.51 90 top
R801  10K  [0402-RES]  26.11,19.51 90 top
R802  10K  [0402-RES]  17.48,9.04 270 top
R803  220R  [0402-RES]  23.06,24.38 90 top
R804  220R  [0402-RES]  25.3,24.38 90 top
R901  10K  [0402-RES]  16.36,9.04 270 top
R902  220R  [0402-RES]  9.35,32.11 180 top
R903  220R  [0402-RES]  9.35,34.54 180 top
R904  220R  [0402-RES]  9.35,36.98 180 top
R905  220R  [0402-RES]  8.94,10.57 180 top
R906  220R  [0402-RES]  8.94,13 180 top
R907  220R  [0402-RES]  8.94,15.44 180 top
R908  220R  [0402-RES]  8.94,17.88 180 top
R909  220R  [0402-RES]  8.94,4.06 180 top
R910  220R  [0402-RES]  8.94,5.18 180 top
R911  220R  [0402-RES]  9.35,33.32 180 top
R912  220R  [0402-RES]  9.35,35.76 180 top
R913  220R  [0402-RES]  9.35,38.2 180 top
R914  220R  [0402-RES]  8.94,11.79 180 top
R915  220R  [0402-RES]  8.94,14.22 180 top
R916  220R  [0402-RES]  8.94,16.66 180 top
R917  220R  [0402-RES]  8.94,19.1 180 top
R918  10K/0.1%  [0402-RES]  13,21.34 270 top
R919  10K/0.1%  [0402-RES]  13,23.37 270 top
R922  10K/0.1%  [0402-RES]  11.07,19.71 180 top
R1001  100K  [0402-RES]  15.65,5.49 180 top
R1002  10K  [0402-RES]  15.24,9.04 90 top
R1101  10K/0.1%  [0402-RES]  59.94,28.35 0 top
R1102  10K/0.1%  [0402-RES]  59.94,29.46 0 top
R1103  1M  [0402-RES]  65.84,25.6 0 top
R1104  1M  [0402-RES]  65.84,26.72 0 top
R1105  453K  [0402-RES]  55.68,36.27 0 top
R1106  56K  [0402-RES]  57.2,35.76 270 top
R1107  105K  [0402-RES]  55.68,35.15 180 top
R1109  453K  [0402-RES]  55.68,33.73 0 top
R1110  56K  [0402-RES]  57.2,33.22 270 top
R1111  105K  [0402-RES]  55.68,32.61 180 top
R1112  453K  [0402-RES]  55.68,31.19 0 top
R1113  56K  [0402-RES]  57.2,30.58 270 top
R1114  105K  [0402-RES]  55.68,30.07 180 top
R1115  0R  [0402-RES]  60.55,36.58 180 top
RN1101  1M  [EXB28V]  56.9,28.04 90 top
S1RX  PAD.04  [PAD.04X.04]  31.7,34.14 270 bottom
S1TX  PAD.04  [PAD.04X.04]  31.7,39.22 0 bottom
S2RX  PAD.04  [PAD.04X.04]  23.98,34.14 270 bottom
S2TX  PAD.04  [PAD.04X.04]  31.7,36.68 90 bottom
S3RX  PAD.04  [PAD.04X.04]  32.11,3.25 270 bottom
S3TX  PAD.04  [PAD.04X.04]  33.73,12.19 0 bottom
S4RX  PAD.04  [PAD.04X.04]  23.98,7.52 45 bottom
S4TX  PAD.04  [PAD.04X.04]  24.38,9.35 45 bottom
S5_RX  PAD.04  [PAD.04X.04]  24.38,2.03 45 bottom
S5_TX  PAD.04  [PAD.04X.04]  23.77,4.57 45 bottom
S601  RESET  [EVQP7J01K]  25.6,38.2 180 top
S801  RESET  [EVQP7J01K]  25.6,2.34 0 top
U101  STM32F4X7VX  [TQFP100]  38.2,19.91 45 top
U102  FM25V01  [SO08]  49.78,28.45 180 top
U201  TXS0108QFN20  [QFN20-RGY]  28.85,30.07 90 top
U202  TXS0108QFN20  [QFN20-RGY]  34.54,3.25 180 top
U301  2908-05WB-MG  [MICROSD]  62.18,18.8 90 bottom
U302  NUF2042XV6  [SOT563-6]  43.89,32.51 180 top
U401  MAX3051  [SOT23-8]  40.23,3.66 0 top
U501  L3GD20  [L3G4200DH-MAN]  64.82,12.8 270 top
U502  L3GD20H  [LGA-16L]  58.52,7.82 270 top
U504  LSM303D  [LGA-16L]  65.13,3.86 180 top
U505  MPU-6000  [QFN-24]  65.74,19.3 270 top
U506  MS5611-01BA  [MS5611-01BA]  65.13,8.03 270 top
U601  BQ24315  [QFN8-DSG]  37.69,36.47 0 top
U602  BQ24315  [QFN8-DSG]  62.59,26.42 90 top
U603  MIC5332  [MLF-8-EPAD]  56.79,14.12 0 top
U701  TCA62724FMG  [SON10]  49.58,14.63 180 top
U702  LT3469  [SOT23-8]  13,28.04 90 top
U703  LRTB GFTG-T7AW-1+V7A7-29+R5T9-49-L  [6-PLCC]  51.61,20.32 90 bottom
U801  STM32F10XCXT6  [TQFP48]  21.95,14.63 225 top
U901  TXS0108QFN20  [QFN20-RGY]  13.41,35.76 180 top
U902  TXS0108QFN20  [QFN20-RGY]  13,15.04 180 top
U903  74LVC2G240  [TSSOP8_SOT505-2]  11.38,1.73 270 top
U1001  BQ24313  [QFN8-DSG]  13.41,5.59 270 top
U1002  MIC5332  [MLF-8-EPAD]  13.41,8.53 90 top
U1101  LTC4417  [MO-220]  61.87,33.32 0 top
U1102  NTHD4102PT1G  [1206-8]  66.45,37.59 270 top
U1103  NTHD4102PT1G  [1206-8]  66.45,33.32 270 top
U1104  NTHD4102PT1G  [1206-8]  66.45,29.06 270 top
VBUS  PAD.04  [PAD.04X.04]  46.23,33.32 270 top
VDD_3V1101  PAD.04  [PAD.04X.04]  40.64,30.89 0 bottom
VDD_5V_BRICK  PAD.04  [PAD.04X.04]  63.91,37.49 270 bottom
VDD_5V_IN  PAD.04  [PAD.04X.04]  54.76,25.3 270 top
VDD_SERVO  PAD.04  [PAD.04X.04]  52.12,39.52 0 top
VDDA_3V1101  PAD.04  [PAD.04X.04]  62.99,1.22 0 bottom
X101  3.2x2.5 mm / 24 MHz / 15 ppm  [OSCILLATOR-3.2X2.5]  29.29,10.18 135 top
X503  0512811094  [51281-1094]  59.13,1.22 180 top
X801  3.2x2.5 mm / 24 MHz / 15 ppm  [OSCILLATOR-3.2X2.5]  16.46,21.54 45 top

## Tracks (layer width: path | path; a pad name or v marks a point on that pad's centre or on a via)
!ACCEL_MAG_CS  (via drill 0.15, 0.2)
  Top 0.152: U101.9 31.92,16.46 v32,16.46 | 64.63,5.28 U504.8 64.63,5.68 64.41,5.89 64.21,5.89 63.91,6.2 63.91,7.62 v63.6,7.92 | X503.6 56.63,2.91 56.08,3.45 v56.08,8.64
  Horizontal 0.152: v32,16.46 32,15.65 33.63,14.02 33.83,14.02 34.24,14.43 35.66,14.43 39.62,10.46 41.25,10.46 42.57,9.14 53.65,9.14 53.95,8.84 55.88,8.84 v56.08,8.64 57.3,8.64 57.51,8.84 58.12,8.84 v58.73,8.23
  Vertical 0.152: v63.6,7.92 63.3,7.92 63.09,7.72 63.09,6.91 62.79,6.6 62.08,6.6 61.67,7.01 59.94,7.01 v58.73,8.23
!BARO_CS  (via drill 0.15, 0.2)
  Top 0.152: v32.82,19.91 33.22,20.32 33.22,24.89 U101.88 | U101.88 | v62.59,7.21 62.87,6.93 U506.5
  Horizontal 0.152: v32.82,19.91 33.83,18.9 44.6,18.9 45.92,17.58 60.55,17.58 61.98,16.15 v61.98,14.12
  Vertical 0.152: v62.59,7.21 62.59,9.86 62.89,10.26 62.89,10.57 62.59,10.87 62.59,13.61 v61.98,14.12
!FMU-LED_AMBER  (via drill 0.2)
  Top 0.152: U101.43 44.7,16.95 v44.7,16.97 | R707.P$1 17.98,37.79 17.37,37.19 17.37,32.92 19,31.29 19,30.79 18.49,30.28 v16.36,30.28
  Horizontal 0.152: v44.7,16.97 43.89,17.78 29.97,17.78 28.04,19.71 28.04,21.13 27.43,21.74 27.03,21.74 26.31,22.45 26.31,22.96 25.7,23.57 23.37,23.57 16.66,30.28 v16.36,30.28
!FRAM_CS
  Top 0.152: U101.57 47.24,24.71 47.24,27.03 49.78,29.57 49.78,32.21 50.09,32.51 51.21,32.51 51.69,32.03 U102.1
!GYRO_CS  (via drill 0.2)
  Top 0.152: U101.7 32.64,18.59 v32.72,18.59 | X503.7 56.13,2.69 v56.08,2.74 | U501.5 62.34,13.78 v61.77,13.21 | U502.5 57.52,9.64 56.9,10.26 v56.9,10.36
  Horizontal 0.152: v32.72,18.59 44.4,18.59 45.72,17.27 56.59,17.27 57.4,16.46 v57.4,12.5 61.06,12.5 v61.77,13.21
  Vertical 0.152: v56.08,2.74 56.08,7.92 55.58,8.43 55.58,9.04 v56.9,10.36 56.9,11.07 57.4,11.58 v57.4,12.5
!IO-LED_AMBER  (via drill 0.2)
  Top 0.152: U801.28 23.37,11.44 v23.37,11.48 | v21.95,7.62 21.95,6.91 22.55,6.3 22.55,5.99 R709.P$1
  Bottom 0.152: v23.37,11.48 23.37,10.16 21.95,8.74 v21.95,7.62
!IO-LED_BLUE
  Top 0.152: U801.27 24.38,9.72 24.38,8.74 24.28,8.64 R712.P$1
!IO-LED_SAFETY
  Top 0.152: U801.26 23.98,9.42 23.98,8.94 23.16,8.13 R710.P$2
!MPU_CS  (via drill 0.2)
  Top 0.152: U101.17 33.98,12.84 34.65,13.51 34.65,13.72 34.85,13.92 v34.85,15.34 | U505.8 63.26,20.05 63.09,20.22 60.25,20.22 v59.84,19.81
  Horizontal 0.152: v34.85,15.34 34.85,15.65 35.36,16.15 41.55,16.15 41.86,16.36 v41.86,16.97 | v41.15,25.6 42.27,26.72 55.17,26.72 55.37,26.52 55.37,24.38 55.17,24.18 55.17,23.37 v55.78,22.76
  Vertical 0.152: v41.86,16.97 41.86,24.89 v41.15,25.6 | v59.84,19.81 56.79,19.81 55.98,20.62 55.98,22.55 v55.78,22.76
!SBUS_OUTPUT_EN  (via drill 0.2)
  Top 0.152: U903.7 12.62,2.05 12.39,1.83 12.39,0.51 12.6,0.3 13.92,0.3 15.24,1.63 15.24,2.23 15.65,2.64 17.17,2.64 17.48,2.95 v17.48,3.56 | v26.11,13.82 24.69,15.24 24.69,15.61 U801.40
  Horizontal 0.152: v26.11,13.82 26.11,11.68 22.96,8.53 22.96,2.54 22.25,1.83 18.29,1.83 17.48,2.74 v17.48,3.56
!SPI_EXT_NSS  (via drill 0.2)
  Top 0.152: U101.3 30.38,19.16 v30.38,19.51
  Horizontal 0.152: v35.87,33.33 42.06,33.33 43.38,32 v52.73,32
  Vertical 0.152: v35.87,33.33 33.93,31.39 33.93,23.37 30.38,19.81 v30.38,19.51
  Bottom 0.15: 53.07,31.67 53.82,31.67 53.95,31.8 54.36,31.8 54.56,31.6 56.74,31.6 J403.5
  Bottom 0.152: 53.07,31.67 v52.73,32
!VBUS_VALID  (via drill 0.2)
  Top 0.152: RN1101.2 57.96,27.79 v58.01,27.74 | U1101.P$9 61.62,30.84 61.16,30.38 60.86,30.38 v60.76,30.28 | U101.15 34.34,14.63 v34.34,15.85
  Horizontal 0.152: v34.34,15.85 34.34,16.05 35.56,17.27 40.95,17.27 v41.25,16.97 | v40.03,25.6 40.64,24.99 41.25,24.99 42.67,26.42 52.12,26.42 !VBUS_VALID.P$1
  Vertical 0.152: !VBUS_VALID.P$1 54.66,25.3 55.17,25.81 55.17,27.53 55.37,27.74 v58.01,27.74 60.35,27.74 60.76,28.14 v60.76,30.28 | v41.25,16.97 41.25,24.38 v40.03,25.6
  other vias: 53.24,25.3
!VDD_5V_HIPOWER_OC  (via drill 0.2)
  Top 0.15: R602.P$1 39.47,32.66 38.41,33.73 v38.41,34.34
  Top 0.152: U101.41 v43.69,16.56 | v38.41,34.34 38.44,34.38 U601.4
  Vertical 0.152: v43.69,16.56 43.69,25.3 40.44,28.55 40.44,31.7 38.41,33.73 v38.41,34.34
!VDD_5V_PERIPH_EN  (via drill 0.2)
  Top 0.152: U101.67 43.28,27.82 v43.28,27.94 | R615.P$1 v61.06,27.23 61.12,27.17 U602.5 | v39.12,34.34 39.12,36.75 U601.5
  Horizontal 0.152: 60.86,27.03 v61.06,27.23 60.45,26.62 58.93,26.62 58.52,26.21 57.51,26.21 55.98,27.74 55.07,27.74 54.86,27.94 51,27.94 50.09,27.03 44.2,27.03 v43.28,27.94
  Vertical 0.152: v43.28,27.94 40.74,30.48 40.74,31.9 39.12,33.53 v39.12,34.34
!VDD_5V_PERIPH_OC  (via drill 0.2)
  Top 0.15: v56.08,24.59 57.1,25.6 R604.P$1
  Top 0.152: U602.4 63.54,27.57 v63.6,27.64 | v46.23,19.3 46.02,19.1 46.02,17.75 U101.46
  Horizontal 0.15: v56.08,24.59 62.38,24.59 63.5,25.7 63.5,27.53 v63.6,27.64
  Horizontal 0.152: v46.94,27.84 50.09,27.84 50.8,28.55 54.76,28.55 55.27,28.04 56.39,28.04 57.51,26.92 58.62,26.92 59.33,27.64 60.66,27.64 60.76,27.74 61.37,27.74 61.47,27.64 v63.6,27.64
  Vertical 0.152: v46.94,27.84 45.82,26.72 45.82,25.81 46.23,25.4 46.23,20.52 45.92,20.22 45.92,19.51 v46.23,19.3
!VDD_BRICK_VALID  (via drill 0.2)
  Top 0.152: U101.91 30.59,25.4 v30.48,25.4 | RN1101.4 57.87,28.92 v58.12,29.16 | U1101.P$7 60.08,31.43 v59.84,31.19 | !VDD_BRICK_VALID.P$1 52.93,26.11 52.43,25.6 52.43,24.99 52.93,24.49 v52.93,24.08
  Horizontal 0.152: v31.19,32.11 33.22,32.11 33.53,31.8 38.2,31.8 39.22,30.79 53.65,30.79 53.85,30.58 54.36,30.58 54.56,30.79 59.44,30.79 v59.84,31.19
  Vertical 0.152: v30.48,25.4 31.19,26.11 v31.19,32.11 | v59.84,31.19 58.12,29.46 v58.12,29.16 57.61,29.67 53.85,29.67 52.93,28.75 52.93,26.01 52.53,25.6 52.53,24.99 52.93,24.59 v52.93,24.08
!VDD_SERVO_VALID  (via drill 0.2)
  Top 0.152: U101.93 31.39,23.18 v31.39,22.76 | RN1101.3 57.96,28.29 v58.22,28.55 | U1101.P$8 61.12,30.95 60.96,30.79 60.35,30.79 v60.25,30.68 | !VDD_SERVO_VALID.P$1 54.36,26.21 v54.05,25.91
  Horizontal 0.152: v31.7,31.6 33.22,31.6 33.33,31.5 36.47,31.5 37.49,30.48 53.44,30.48 53.75,30.18 54.46,30.18 54.76,30.48 59.64,30.48 59.84,30.68 v60.25,30.68
  Vertical 0.152: v31.39,22.76 31.7,23.06 v31.7,31.6 | v54.05,25.91 53.34,26.62 53.34,28.25 53.65,28.55 v58.22,28.55 58.52,28.55 58.73,28.75 60.05,28.75 60.25,28.96 v60.25,30.68
ACCEL_DRDY  (via drill 0.2)
  Top 0.152: U504.11 63.2,3.86 v62.99,4.06 | v31.9,18.59 31.9,20.32 32.61,21.03 32.61,24.08 U101.90 | v58.12,2.85 58.12,1.24 X503.3
  Horizontal 0.152: v62.99,4.06 59.33,4.06 v58.12,2.85 57.2,1.93 48.97,1.93 47.24,3.66 44.09,3.66 43.89,3.66 39.01,3.66 36.17,6.5 v32.72,6.5
  Vertical 0.152: v31.9,18.59 33.02,17.48 33.02,6.81 v32.72,6.5
ALARM  (via drill 0.2)
  Top 0.152: U101.77 37.34,28.55 v38.41,28.55 | R701.P$2 8.85,28.34 v9.35,27.84
  Horizontal 0.152: v38.41,28.55 32.51,28.55 28.65,32.41 16.97,32.41 15.14,34.24 10.06,34.24 9.35,33.53 v9.35,27.84
BATT_CURRENT_SENS  (via drill 0.2)
  Top 0.152: U101.26 40.03,9.6 v40.03,9.04 | v59.03,28.25 59.13,28.35 R1101.P$1
  Horizontal 0.152: v38.91,27.84 39.52,28.45 50.19,28.45 50.7,28.96 54.86,28.96 55.47,28.35 56.59,28.35 57.71,27.23 58.42,27.23 58.62,27.43 58.62,27.84 v59.03,28.25
  Vertical 0.152: v40.03,9.04 40.03,10.06 38.81,11.28 38.81,23.67 39.32,24.18 39.32,27.43 v38.91,27.84
BATT_CURRENT_SENS_PROT  (via drill 0.2)
  Top 0.152: v63.6,28.35 L1101.P$1 | R1104.P$1 v64.62,26.72
  Vertical 0.152: v64.62,26.72 64.62,27.33 v63.6,28.35
  Bottom 0.152: J601.3 65.72,34.15 66.14,33.73 66.14,29.46 65.02,28.35 v63.6,28.35
BATT_VOLTAGE_SENS  (via drill 0.2)
  Top 0.152: U101.25 37.14,10.36 v37.8,10.36 | v58.93,29.46 R1102.P$1
  Horizontal 0.152: v37.69,29.87 37.9,30.07 53.34,30.07 53.54,29.87 54.66,29.87 54.86,30.07 58.32,30.07 v58.93,29.46
  Vertical 0.152: v37.8,10.36 36.88,11.28 36.88,26.11 37.69,26.92 v37.69,29.87
BATT_VOLTAGE_SENS_PROT  (via drill 0.2)
  Top 0.152: L1102.P$1 63.39,29.36 v63.6,29.36 | R1103.P$1 v64.62,25.6
  Vertical 0.152: v64.62,25.6 65.13,26.11 65.13,27.84 v63.6,29.36
  Bottom 0.152: J601.4 65.45,32.9 65.84,32.51 65.84,29.67 65.53,29.36 v63.6,29.36
CAN1_RX  (via drill 0.2)
  Top 0.152: v36.17,26.92 36.14,26.92 U101.81 | U401.4 41.7,2.48 v42.16,2.95
  Horizontal 0.152: v42.16,2.95 38.91,2.95 v38.2,3.66
  Vertical 0.152: v38.2,3.66 36.58,5.28 36.58,26.52 v36.17,26.92
CAN1_TX  (via drill 0.2)
  Top 0.152: v35.46,26.92 35.43,26.92 U101.82 | U401.1 38.66,2.48 v38.2,2.95
  Vertical 0.152: v35.46,26.92 36.27,26.11 36.27,4.88 v38.2,2.95
CAN2_RX
  Top 0.152: U101.51 49.13,22.36 R216.P$1
CAN2_TX
  Top 0.152: U101.92 30.39,24.89 30.07,24.89 29.87,25.09 R215.P$1
CAN_H  (via drill 0.2)
  Top 0.152: U401.7 39.91,5.61 39.52,5.99 v39.52,6.3 v39.53,6.31 R409.P$1
  Bottom 0.152: CAN_H.P$1 v39.52,6.3 39.93,6.71 40.44,6.71 40.83,6.32 J405.2
CAN_L  (via drill 0.2)
  Top 0.152: U401.6 40.56,5.77 v40.23,6.1 40.53,6.39 R409.P$2
  Bottom 0.152: J405.3 40.42,5.07 | 40.42,5.07 CAN_L.P$1 | 40.42,5.07 40.42,5.91 v40.23,6.1
FMU-!RESET  (via drill 0.2)
  Top 0.15: U603.3 55.62,13.87 v55.27,13.51
  Top 0.152: v49.07,15.24 49.07,16 U701.4 | v33.73,14.73 U101.14 | S601.A1 28.85,37.48 C609.P$2 29.36,37.19 v29.36,36.27 | v52.32,13.51 52.32,13.11 52.53,12.9 53.13,12.9 53.14,12.9 R635.P$1
  Horizontal 0.152: v27.53,20.93 27.53,19.71 30.58,16.66 31.5,16.66 31.8,16.97 32.41,16.97 32.72,16.66 32.72,15.75 v33.73,14.73 48.56,14.73 v49.07,15.24 49.17,15.34 50.49,15.34 v52.32,13.51 v55.27,13.51
  Vertical 0.152: v27.53,20.93 29.36,22.76 v29.36,36.27
FMU-BOOT0  (via drill 0.2)
  Top 0.152: U101.94 29.49,24.38 R611.P$2 27.42,25.41 v27.23,25.6
  Bottom 0.152: FMU-BOOT1101.P$1 26.82,25.6 v27.23,25.6
FMU-CH1  (via drill 0.2)
  Top 0.152: v45.72,20.73 45.72,17.34 U101.45 | U901.7 16.32,36.51 17.07,35.76 17.07,32.51 v18.49,31.09
  Horizontal 0.152: v45.72,20.73 45.52,20.93 35.56,20.93 31.6,24.89 24.08,24.89 18.49,30.48 v18.49,31.09
FMU-CH1-PROT
  Top 0.406: R913.P$2 7.34,38.2 J901.46
FMU-CH2  (via drill 0.2)
  Top 0.152: U101.44 45.21,17.15 v45.21,20.32 | U901.6 16.11,36.01 16.76,35.36 16.76,32.11 v17.78,31.09
  Horizontal 0.152: v45.21,20.32 44.91,20.62 35.36,20.62 31.39,24.59 23.88,24.59 17.78,30.68 v17.78,31.09
FMU-CH3  (via drill 0.2)
  Top 0.152: U101.42 44.2,16.75 v44.2,19.81 | U901.5 15.9,35.51 16.46,34.95 16.46,31.7 v17.07,31.09
  Horizontal 0.152: v44.2,19.81 43.69,20.32 35.15,20.32 31.19,24.28 23.67,24.28 17.07,30.89 v17.07,31.09
FMU-CH4  (via drill 0.2)
  Top 0.152: U101.40 43.18,16.35 v43.18,19.81 | U901.4 15.89,35.01 16.15,34.75 16.15,31.29 v16.36,31.09
  Horizontal 0.152: v43.18,19.81 35.15,19.81 31.09,23.88 23.57,23.88 v16.36,31.09
FMU-CH5  (via drill 0.2)
  Top 0.152: U101.60 44.28,23.88 v42.57,23.88 | v15.65,31.6 15.85,31.8 15.85,34.34 15.68,34.51 U901.3
  Horizontal 0.152: v42.57,23.88 42.16,23.47 36.58,23.47 28.25,31.8 15.85,31.8 v15.65,31.6
FMU-CH6  (via drill 0.2)
  Top 0.152: U101.61 43.88,24.18 43.18,24.18 v42.98,24.38 | U901.1 15.16,32.51 v15.24,32.51
  Horizontal 0.152: v42.98,24.38 42.27,24.38 41.66,23.77 36.78,23.77 28.45,32.11 15.65,32.11 v15.24,32.51
FMU-CH6-PROT
  Top 0.406: R902.P$2 8.53,32.11 8.23,31.8 8.23,30.18 7.72,29.67 7.72,27.96 J901.31
FMU-I2C1_SCL  (via drill 0.2)
  Top 0.152: U101.95 31.09,22.08 v31.09,22.05 | R404.P$1 R401.P$1 v43.98,2.63 v43.99,2.64
  Horizontal 0.152: v43.99,2.64 43.18,2.64 42.47,1.93 35.66,1.93 35.46,1.73 32.41,1.73 31.9,2.23 31.29,2.23 v30.79,1.73
  Vertical 0.152: v31.09,22.05 30.48,22.66 29.87,22.66 28.04,20.83 28.04,4.47 v30.79,1.73
FMU-I2C1_SDA  (via drill 0.2)
  Top 0.152: U101.96 30.48,21.98 v30.48,21.95 | R405.P$1 R402.P$1 43.38,0.3 42.57,0.3 42.27,0.61 v42.27,1.22
  Horizontal 0.152: v42.27,1.22 41.66,0.61 32.72,0.61 v31.6,1.73
  Vertical 0.152: v30.48,21.95 30.18,22.25 29.97,22.25 28.35,20.62 28.35,4.98 v31.6,1.73
FMU-I2C2_SCL
  Top 0.152: U701.3 R306.P$1 49.49,16.98 49.17,16.66 47.82,16.66 U101.47
FMU-I2C2_SDA
  Top 0.152: U701.2 50.08,16.26 R307.P$1 50.69,16.98 50.19,17.48 48.87,17.48 48.56,17.17 48.02,17.17 U101.48
FMU-SWCLK  (via drill 0.2)
  Top 0.152: U101.76 37.08,30.11 v37.08,30.18
  Bottom 0.152: JX301.4 32.97,20.57 32.72,20.83 32.72,22.35 33.73,23.37 33.73,27.94 35.97,30.18 v37.08,30.18
FMU-SWDIO  (via drill 0.2)
  Top 0.152: v39.73,27.94 39.86,27.94 U101.72
  Bottom 0.152: v39.73,27.94 38.41,29.26 35.56,29.26 34.04,27.74 34.04,23.37 34.54,22.86 JX301.2
FMU-SWO  (via drill 0.2)
  Top 0.152: v32.41,19.3 32.31,19.41 32.31,20.22 32.92,20.83 32.92,24.49 U101.89
  Bottom 0.152: v32.41,19.3 JX301.6
FMU-UART4_RX
  Top 0.152: U101.24 35.66,9.6 35.66,8.74 36.27,8.13 36.27,5.99 36.98,5.28 36.98,4.67 36.81,4.5 U202.8
FMU-UART4_TX
  Top 0.152: U101.23 35.36,10 35.36,8.53 35.97,7.92 35.97,5.33 U202.9
FMU-UART7_RX  (via drill 0.2)
  Top 0.152: U202.4 35.52,2.5 v35.26,2.23 | U101.38 42.88,15.24 v42.67,15.24
  Horizontal 0.152: v35.46,15.24 v42.67,15.24
  Vertical 0.152: v35.26,2.23 35.5,2.23 35.87,2.6 35.87,3.25 34.65,4.47 34.65,9.55 35.66,10.57 35.66,15.04 v35.46,15.24
FMU-UART7_TX  (via drill 0.2)
  Top 0.152: 44.19,14.63 U101.39 45.01,13.81 v45.01,13.51 | U202.5 v35.31,3
  Horizontal 0.152: v35.31,3 36.08,2.23 42.16,2.23 43.08,3.15 v44.5,3.15
  Vertical 0.152: v44.5,3.15 44.5,10.67 45.01,11.18 v45.01,13.51
FMU-UART8_RX  (via drill 0.2)
  Top 0.152: U202.6 34.79,3.5 34.54,3.25 v34.54,2.95 | U101.97 30.38,21.37 v30.38,21.34
  Vertical 0.152: v34.54,2.95 31.8,2.95 28.96,5.79 28.96,19.61 30.38,21.03 v30.38,21.34
FMU-UART8_TX  (via drill 0.2)
  Top 0.152: U202.7 36.23,4.06 34.14,4.06 33.73,3.66 v33.73,2.44 | v29.77,21.23 29.77,21.27 U101.98
  Vertical 0.152: v33.73,2.44 31.7,2.44 28.65,5.49 28.65,20.12 v29.77,21.23
FMU-USART2_CTS
  Top 0.152: U201.9 32.62,28.32 U101.84
FMU-USART2_RTS
  Top 0.152: U101.85 32.6,27.64 30.28,27.64 30.1,27.81 U201.8
FMU-USART2_RX
  Top 0.152: U101.87 31.8,27.03 29.67,27.03 29.1,27.59 U201.6
FMU-USART2_TX
  Top 0.152: U101.86 32.2,27.33 29.97,27.33 29.6,27.7 U201.7
FMU-USART3_CTS  (via drill 0.2)
  Top 0.152: U101.58 44.91,23.08 v44.91,22.96 | v27.64,26.52 27.6,26.55 U201.3
  Horizontal 0.152: v44.91,22.96 43.79,21.84 36.17,21.84 31.29,26.72 27.84,26.72 v27.64,26.52
FMU-USART3_RTS  (via drill 0.2)
  Top 0.152: U101.59 44.48,23.37 v43.08,23.37 | v25.91,29.77 26.35,29.32 U201.1
  Horizontal 0.152: v43.08,23.37 42.88,23.16 36.37,23.16 29.77,29.77 v25.91,29.77
FMU-USART3_RX  (via drill 0.2)
  Top 0.152: U101.56 45.52,22.28 v45.52,22.25 | v28.14,26.11 28.1,26.15 U201.4
  Horizontal 0.152: v45.52,22.25 44.81,21.54 35.97,21.54 31.09,26.42 28.45,26.42 v28.14,26.11
FMU-USART3_TX  (via drill 0.2)
  Top 0.152: U101.55 45.72,21.77 v45.72,21.64 | v28.85,25.91 28.6,26.16 U201.5
  Horizontal 0.152: v45.72,21.64 45.31,21.23 35.76,21.23 31.09,25.91 v28.85,25.91
FMU-VDD_3V3  (via drill 0.2, 0.3)
  Top 0.15: R604.P$2 56.09,25.61 55.47,24.99 55.47,24.18 v55.78,23.88
  Top 0.25: v39.83,31.29 39.83,31.8 R602.P$2
  Top 0.254: 15.14,34.04 U901.2 15.16,33.55 v15.04,33.43 | U101.11 30.69,13.82 v30.48,13.82 29.57,13.82 C610.P$1 | U101.22 34.76,10.11 C612.P$1 34.65,9.95 34.65,7.72 35.04,7.32 C202.P$1 35.29,6.66 U202.10 | C101.P$1 41.34,9.7 U101.28 39.46,11.58 v39.42,11.58 36.92,11.58 36.58,11.92 36.51,11.86 | C402.P$1 41.45,1.22 v41.55,1.32 42.27,2.03 R401.P$2 R402.P$2 | U401.3 40.56,1.39 C402.P$1 | C402.P$1 40.73,0.91 40.23,0.41 37.39,0.41 U202.2 36.27,1.52 35.76,1.52 35.56,1.73 33.53,1.73 33.3,1.5 U202.19 | U101.50 48.3,18.69 49.58,18.69 | 49.58,18.69 50.39,18.69 | v48.36,19.1 48.36,18.76 U101.50 | 48.15,18.5 U101.50 | v11.79,33.43 11.66,33.55 U901.19 | C201.P$1 31.86,29.32 U201.10 | v51.71,24.38 51.71,25.81 U102.8 U102.7 | U102.3 49.15,29.84 v48.77,29.46 47.9,28.6 R304.P$2 R305.P$2 | C201.P$1 32.52,29.57 R303.P$2 R302.P$2 R301.P$2 | v33.02,29.26 32.42,29.26 C201.P$1 | R306.P$2 49.58,18.69 | R307.P$2 50.8,18.29 50.39,18.69 | U101.75 40.59,30.79 C606.P$1 40.34,31.29 v39.83,31.29 | U101.22 36.51,11.86 | U101.21 U101.22 | U101.19 35.53,13.01 36.51,12.03 36.51,11.86 | U101.100 27.18,22.45 v27.13,22.45 26.61,22.45 C608.P$1 | v26.42,27.94 26.8,28.32 U201.2 27.13,28.35 27.13,28.85 27.33,29.06 27.33,31.09 27.1,31.32 U201.19 26.09,31.82 25.7,32.21 D2.A | C607.P$1 51.21,19.51 50.39,18.69 | U701.10 51,13.68 51,15.65 | 51,15.65 50.64,16 U701.1 | 51,15.65 C701.P$1 52.42,15.64 v52.43,15.65 | C902.P$1 14.16,39.07 U901.10 14.54,38.01 v14.73,38.2
  Bottom 0.254: VDD_3V1101.P$1 40.64,30.99 C606.P$1 40.08,31.04 v39.83,31.29 | v14.73,38.2 15.04,37.9 v15.04,33.43
  Bottom 0.406: v11.79,33.43 v15.04,33.43 | JX301.1 v38.61,24.38 | U301.4 66,20.16 66.24,19.91 66.24,15.14 65.84,14.73 59.03,14.73 v58.62,14.33
  pour Power: 28.85,1.32 28.85,17.07 21.13,24.79 14.12,24.79 14.12,33.73 42.67,33.73 42.67,30.68 58.72,30.68 58.72,1.32
  pour Top (isolate 0.254, rank 2, no thermals): 57.3,14.63 58.42,14.63 58.52,14.73 58.52,14.94 58.72,15.14 59.54,15.14 59.64,15.04 59.64,11.18 59.44,10.97 58.72,10.97 58.52,11.18 58.52,14.02 58.42,14.12 57.3,14.12
FMU-VDD_5V5
  pour Top (isolate 0.254, rank 2, no thermals): 53.04,15.34 56.08,15.34 56.39,15.04 56.39,12.7 56.08,12.4 52.83,12.4 52.53,12.7 52.53,15.04 52.83,15.34
FMU_AUX_ADC1  (via drill 0.2)
  Top 0.152: R408.P$1 37.7,8.95 v37.59,8.84 | v35.15,13.51 35.15,13.33 U101.18
  Bottom 0.152: v37.59,8.84 35.15,11.28 v35.15,13.51
FMU_AUX_ADC1_PROT  (via drill 0.2)
  Top 0.152: R408.P$2 38.7,10.07 v38.61,10.16
  Bottom 0.152: J404.4 45.24,19.07 46.02,18.29 46.02,14.33 45.82,14.12 43.08,14.12 39.12,10.16 v38.61,10.16
FMU_AUX_ADC2
  Top 0.152: U101.33 43.25,11.33 R407.P$1
FMU_AUX_ADC2_PROT  (via drill 0.2)
  Top 0.152: 44.3,10.57 R407.P$2 44.5,10.88 v44.5,11.58
  Bottom 0.152: v44.5,11.58 46.33,13.41 46.33,18.49 43.25,21.57 J404.2
FRAM_MISO
  Top 0.152: U101.53 48.46,23.1 48.46,27.13 50.42,29.08 U102.2
FRAM_MOSI
  Top 0.152: U101.54 47.88,23.23 U102.5
FRAM_SCK
  Top 0.152: U101.52 48.77,22.7 48.77,23.98 49.15,24.36 U102.6
GND  (via drill 0.2, 0.3)
  Top 0.15: v55.07,14.12 55.27,14.33 55.95,14.33 U603.2 | C1101.P$2 69.12,39.25 v69.39,39.52 | C1110.P$2 58.23,30.08 57.61,29.46 55.78,29.46 v55.47,29.16
  Top 0.152: C1107.P$2 65.23,31.5 65.53,31.8 66.34,31.8 66.65,32.11 v66.65,32.72 | C1106.P$2 65.23,35.77 65.53,36.07 65.94,36.07 v66.34,36.47 | C615.P$2 52.93,13.82 v52.63,14.12 | 16.26,5.58 16.26,5.59 | C1108.P$2 58.82,35.26 v58.83,35.26 | C1109.P$2 v58.72,32.72 v58.73,32.72 | L402.P$3 L402.P$5 L402.P$4 | L1102.P$3 L1102.P$5 L1102.P$4
  Top 0.2: v63.2,16.15 C514.P$2 | C512.P$2 v62.38,17.07 | U505.1 66.98,22.02 v66.95,22.05 | v69.49,21.13 69.49,20.42 69.23,20.16 C515.P$2 | U505.18 66.98,16.57 C513.P$2 | C1003.P$2 10.63,8.39 v10.57,8.33
  Top 0.25: C1005.P$2 16.26,4.78 16.26,5.58 R1001.P$1 | 16.26,5.59 16.26,6.81 16.76,7.32 17.37,7.32 | 33.77,10.94 34.17,10.94 U101.20 | 33.78,10.55 33.78,10.92 33.77,10.94 | 33.77,10.94 v33.73,10.97 | C1004.P$2 v13.51,11.18 13.61,11.27 C1002.P$2 | v58.22,3.86 58.32,3.86 | v58.83,5.69 59.03,5.89 U502.12 | v61.98,9.35 61.36,9.35 | 61.46,8.32 C505.P$2 C503.P$2 61.36,9.35 | v65.73,10.06 65.75,10.04 U506.2 U506.3 | 61.27,9.35 61.36,9.35 | C1008.P$2 9.05,9.03 9.14,8.94 v9.45,8.94
  Top 0.254: U501.10 U501.11 U501.12 65.8,10.97 66.65,10.97 66.65,11.18 | U501.10 U501.9 | 64.52,9.14 U506.3 | U504.13 U504.12 65.32,3.36 v65.43,3.25 | U504.5 66.13,4.86 65.43,4.17 v65.43,3.25 | C502.P$2 C504.P$2 69.18,11.79 | 65.8,9.17 U506.2 | 64.52,10.88 U501.10 | v65.43,3.25 65.63,3.06 U504.16 65.63,2.04 66.28,1.39 C509.P$2 | U504.10 64.32,4.36 v65.43,3.25 | R702.P$2 8.13,27.23 v8.13,25.4 8.13,24.79 C703.P$2 | R706.P$2 10.35,31.39 C704.P$2 11.07,32 v10.97,32.11 | U801.47 23.03,18.9 22.76,18.9 21.45,20.21 C803.P$2 | C803.P$2 21.39,20.67 | v20.32,20.73 C803.P$2 | 63.84,10.9 U501.9 | U501.9 63.85,10.97 62.99,10.97 62.99,11.83 U501.8 | 66.65,11.18 66.65,11.83 U501.13 66.76,11.79 69.18,11.79 | U801.35 27.43,12.33 v27.43,12.29 28.38,12.29 X101.2 30.21,12.65 C102.P$2 | C804.P$2 C610.P$2 29.57,15.13 v30.07,14.63 30.8,14.63 U101.10 | 33.78,10.55 C612.P$2 | C103.P$1 32.21,10.97 v33.73,10.97 | U101.27 41.34,8.99 | 41.34,8.99 C101.P$2 | v38.91,1.32 39.01,1.22 C402.P$2 39.91,1.39 U401.2 39.93,2.48 39.93,3.66 | v32.61,5.79 32.9,5.5 U202.11 33.79,6.66 C202.P$2 33.33,6.91 D203.A 32.87,7.57 L203.P$3 | U201.11 31.86,30.82 C201.P$2 32.62,31.09 v32.82,31.09 | U102.4 47.85,31.04 v47.85,29.46 | 40.98,38.56 J301.GND4 | 45.98,38.56 J301.GND1 | 42.3,36.21 J301.GND 41.48,36.21 J301.GND3 | v18.9,16.15 18.9,16.62 U801.8 17.28,18.24 C806.P$1 | D901.A D902.A 11.47,5.58 11.73,5.84 U1001.2 13.26,5.84 | v12.19,16.26 12.26,16.32 U902.11 12.32,17.29 C903.P$2 13.32,19.6 X801.4 15.08,21.79 R919.P$1 | v20.32,20.73 20.32,21.63 D701.A D801.A | U801.23 21.06,10.57 v21.54,10.57 22.45,9.66 C802.P$2 | R704.P$1 51.61,12.51 v51.61,13.41 51.71,13.51 C701.P$2
  Top 0.254: D202.A 23.98,34.23 L202.P$3 L202.P$5 L202.P$4 | C606.P$2 41.75,31.29 | 41.75,31.29 v41.86,31.29 42.11,31.29 C613.P$2 | D404.A 37.08,7.32 L403.P$4 L403.P$5 L403.P$3 | 41.75,31.29 41.75,31.24 U101.74 | R801.P$2 R713.P$2 27.54,20.32 28.85,20.32 29.26,20.73 29.26,21.08 U101.99 27.84,22.5 v27.84,22.66 27.24,23.26 C608.P$2 R611.P$1 | U401.5 41.21,3.66 39.93,3.66 | U401.8 39.26,3.66 39.93,3.66 | U302.2 v43.89,33.73 | v41.05,8.53 41.05,8.7 41.34,8.99 | R102.P$2 45.92,12.3 D403.A 46.24,13.32 L404.P$4 L404.P$5 L404.P$3 48.16,14.43 48.16,15.24 48.58,15.66 U701.5 | X801.2 19.15,20.4 | 19.15,20.4 C805.P$2 | 19.15,20.4 19.47,20.73 v20.32,20.73 | X101.4 29.55,8.72 L203.P$4 | L203.P$4 | L203.P$4 L203.P$5 | L401.P$4 L401.P$5 L401.P$3 62.16,2.24 D401.A | L603.P$3 L603.P$5 L603.P$4 | v67.26,11.18 66.65,11.18 | U502.9 U502.10 U502.11 U502.12 U502.13 | C503.P$2 61.37,9.35 | U903.4 10.12,0.75 v10.16,0.71 | U903.1 10.12,2.7 v10.16,2.74 | C901.P$2 14.36,4.41 U1001.5 U1001.6 13.56,5.34 U1001.P$3 | 17.48,7.28 v17.48,7.32 R802.P$2 | U1001.P$2 13.26,5.84 | U1002.2 13.16,8.38 v13.01,8.53 11.42,8.53 C1003.P$2 | R1002.P$1 v13.82,8.53 | v48.67,20.73 49.01,21.07 C611.P$2 50.7,21.07 | 50.7,21.07 51.16,21.07 C607.P$2 | R610.P$2 50.6,21.16 50.7,21.07 | U702.4 15.71,29.02 v15.75,29.06 15.75,30.52 C702.P$2 | 13.26,5.84 U1001.GND | C801.P$1 25.29,4.38 25.6,4.06 v25.6,1.73 25.49,1.61 S801.B3 21.96,1.61 21.45,2.13 R708.P$1 19.41,2.13 v18.9,2.64 | L201.P$3 L201.P$5 L201.P$4 35.04,36.78 D201.A | L901.P$4 L901.P$5 L901.P$3 10.96,22.77 D903.A | R711.P$1 C902.P$2 12.91,38.26 U901.11 12.85,38.2 v13.31,38.2 | L1101.P$4 L1101.P$5 L1101.P$3
  Top 0.254: U1101.P$10 62.12,32.36 v62.18,32.41 61.87,32.72 U1101.P$25 | 40.03,38.51 R617.P$2 37.94,37.95 U601.6 37.94,36.62 U601.P$3 | U601.2 37.44,36.32 U601.P$2 U601.GND | R615.P$2 R616.P$2 59.44,25.39 v59.74,25.09 | U602.6 62.44,26.67 U602.P$3 | U602.2 62.74,26.17 | 62.74,26.17 U602.P$2 | C609.P$1 27.63,38.7 S601.B3 | 62.74,26.17 62.74,26.27 U602.GND | 69.18,11.79 C508.P$2 69.09,10.88 R403.P$1 68.47,9.95 68.28,9.75 68.28,8.13 | 68.28,8.13 68.48,7.92 C401.P$2 | v67.97,7.52 68.28,7.82 68.28,8.13 | X503.2 58.63,3.45 v58.22,3.86 | C506.P$2 69.22,1.9 v69.19,1.93 v69.18,1.94 C507.P$2 | B601.2 24.07,27.52 v24.08,27.53
  Top 0.4: C1105.P$2 v64.72,39.73
  Top 0.406: J301.GND3 40.98,38.56 | 45.98,38.56 J301.GND2 46.83,35.87 v47.14,35.87 | U1002.GND v13.01,8.53 | C1001.P$2 17.37,7.32 v17.48,7.32 | 40.03,38.51 J301.GND4 | 61.1,16.26 61.1,16.76 | C501.P$2 61.1,18.75 | C602.P$1 v55.27,11.18 | R1115.P$1 v61.57,36.58
  Bottom 0.254: 64.65,4.03 J402.3 65.06,4.03 | v20.83,25.2 20.22,25.81 J801.P$2 | J203.6 34.14,3.7 | J404.5 41.71,17.88 | J302.4 41.86,32.78 | 34.07,30.68 J201.6 | JX801.3 17.78,1.52 | 55.48,29.17 v55.47,29.16 | GND..P$1 38.4,36.17 U601.P$3 | v58.22,3.86 58.17,3.81 J401.4
  Bottom 0.381: v40.44,16.76 40.44,17.88 | J404.3 40.74,20.32 40.44,20.02 40.44,19.51 | JX301.5 40.44,19.3
  Bottom 0.406: JX301.3 JX301.5 | 41.71,17.88 40.44,17.88 40.44,19.3 40.44,19.51 | v40.44,16.76 JX301.9 | J204.6 26.33,2.45 v25.6,1.73 | JX802.3 JX802.5 11.89,20.12 12.19,20.42 12.19,22.35 11.89,22.66 JX802.9 10.57,23.06 L901.P$5 | 41.86,32.78 v41.86,31.29 | v63.8,22.35 v63.8,22.36 U301.6 | J701.2 18.58,15.02 18.9,15.34 v18.9,16.15 | J405.4 40.59,3.81 38.91,2.13 v38.91,1.32 | J203.6 33.1,3.78 32.61,4.27 v32.61,5.79 | v65.43,3.25 65.43,3.66 65.06,4.03 | 17.78,1.52 v18.9,2.64 | J403.7 55.48,29.17
  Bottom 0.61: 34.07,30.68 33.22,30.68 v32.82,31.09 32.34,30.61 J202.6
  other vias: 25.3,27.53 22.76,27.53 62.79,32.41 61.57,32.41 66.95,26.62 68.78,39.52 56.79,14.53 56.79,13.72 57.91,22.66 56.79,23.77 69.39,30.89 68.88,30.89 69.19,23.47 68.68,23.47 67.56,23.88 68.17,23.47 67.56,23.37 61.47,15.44 60.96,15.44 60.55,19.61 61.06,19.61 52.32,29.57 52.32,33.02 30.68,39.93 32.41,39.93 53.44,15.95 53.95,15.95 53.95,16.46 53.44,16.46 69.29,17.48 68.68,17.48
  pour Ground (no thermals): 69.9,40.54 0,40.54 0,0.02 arc90 0.02,0 53,0 53,9.75 61.37,9.75 61.37,23.16 68.68,23.16 68.68,22.35 62.18,22.35 62.18,9.25 53.55,9.25 53.55,0 69.9,0
  pour Bottom (no thermals): 7.72,3.66 7.72,15.04 17.88,15.04 17.88,3.66
  pour Bottom (no thermals): 65.33,30.18 60.76,30.18 60.76,32.61 63.2,32.61 63.2,31.9 65.33,31.9
  pour Bottom (no thermals): 0.41,40.23 2.13,40.23 2.13,0.3 0.41,0.3
  pour Top (no thermals): 0.41,40.23 2.13,40.23 2.13,0.2 0.41,0.2
  pour Bottom (isolate 0.254, rank 4, no thermals): 55.98,13.41 55.98,14.63 56.39,15.04 56.59,28.75 68.28,28.75 68.28,14.73 58.32,14.63 57.81,14.12 57.81,13.61 57.61,13.41
  pour Bottom (no thermals): 35.15,30.78 35.15,40.34 45.42,40.34 45.42,30.78
  pour Top (isolate 0.254, rank 6, no thermals): 56.49,23.98 56.49,22.35 56.59,22.25 58.01,22.25 58.12,22.35 58.12,23.98 58.01,24.08 56.59,24.08
  pour Top (no thermals): 68.17,31.8 69.6,31.8 69.6,29.87 68.17,29.87
  pour Top (isolate 0.254, no thermals): 66.14,27.13 67.06,27.13 67.26,26.92 67.26,25.4 67.06,25.2 66.14,25.2 65.94,25.4 65.94,26.92
  pour Top (isolate 0.254, rank 2, no thermals): 66.14,24.79 69.7,24.79 69.8,24.69 69.8,22.86 69.7,22.76 66.14,22.76 66.04,22.86 66.04,24.69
